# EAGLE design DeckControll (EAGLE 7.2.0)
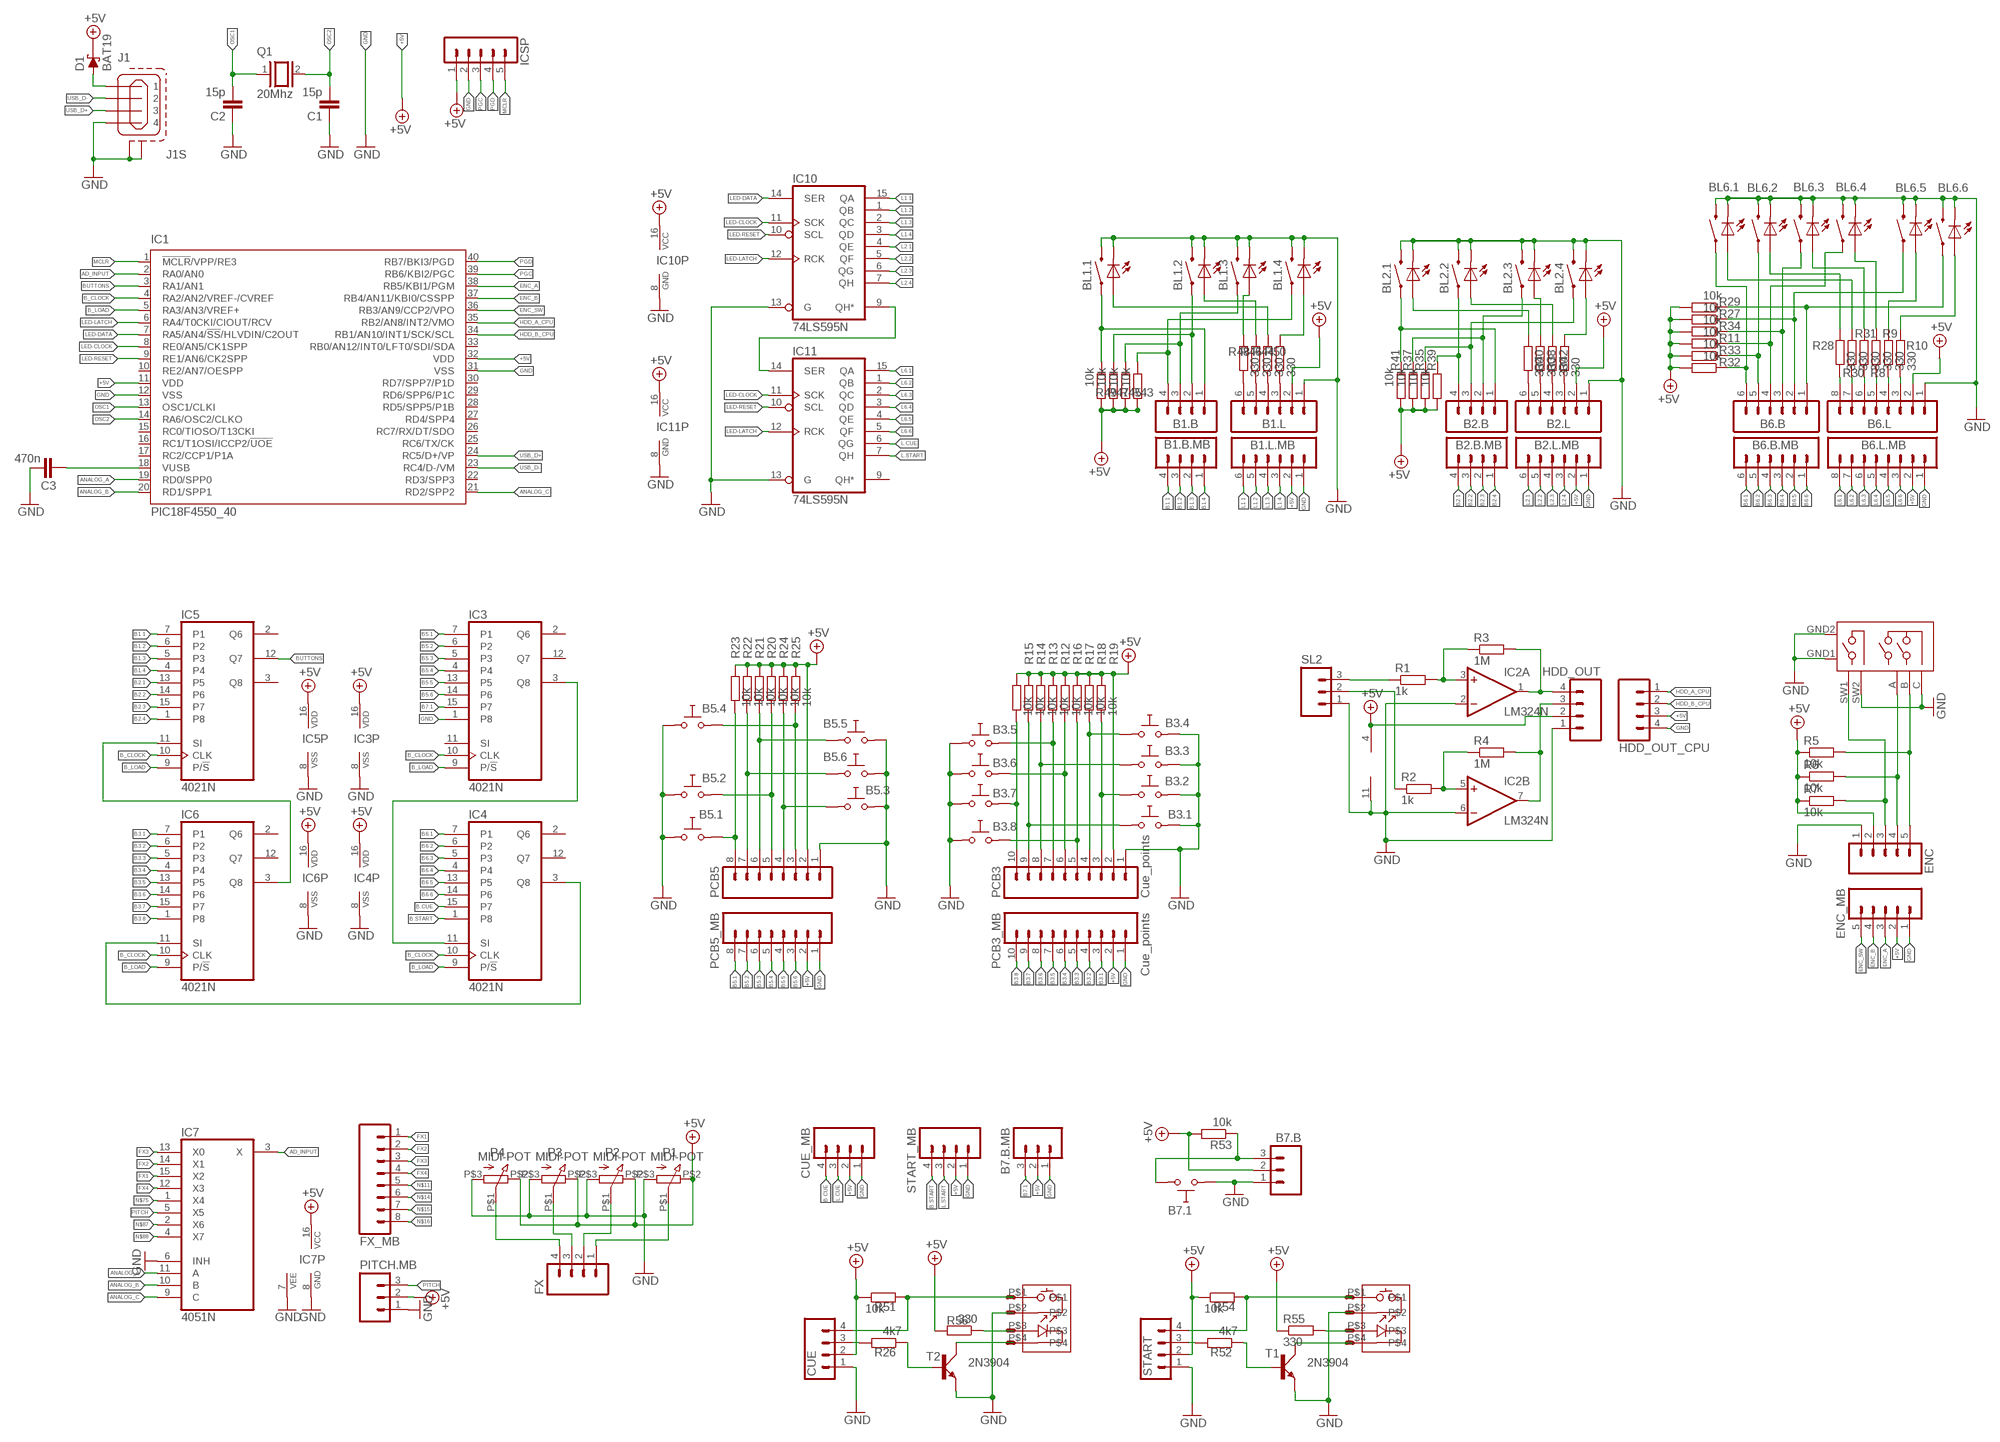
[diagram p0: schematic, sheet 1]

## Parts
ARC01  ARCADE+BTN  [ARCADE_BTN]
ARC02  ARCADE+BTN  [ARCADE_BTN]
B1.B  M04  [04P]
B1.B.MB  M04  [04P]
B1.L  M06  [06P]
B1.L.MB  M06  [06P]
B2.B  M04  [04P]
B2.B.MB  M04  [04P]
B2.L  M06  [06P]
B2.L.MB  M06  [06P]
B3.1  SW-TAKTSS  [SW_TAKT12X12SS]
B3.2  SW-TAKTSS  [SW_TAKT12X12SS]
B3.3  SW-TAKTSS  [SW_TAKT12X12SS]
B3.4  SW-TAKTSS  [SW_TAKT12X12SS]
B3.5  SW-TAKTSS  [SW_TAKT12X12SS]
B3.6  SW-TAKTSS  [SW_TAKT12X12SS]
B3.7  SW-TAKTSS  [SW_TAKT12X12SS]
B3.8  SW-TAKTSS  [SW_TAKT12X12SS]
B5.1  SW-TAKTSS  [SW_TAKT12X12SS]
B5.2  SW-TAKTSS  [SW_TAKT12X12SS]
B5.3  SW-TAKTSS  [SW_TAKT12X12SS]
B5.4  SW-TAKTSS  [SW_TAKT12X12SS]
B5.5  SW-TAKTSS  [SW_TAKT12X12SS]
B5.6  SW-TAKTSS  [SW_TAKT12X12SS]
B6.B  M06  [06P]
B6.B.MB  M06  [06P]
B6.L  M08  [08P]
B6.L.MB  M08  [08P]
B7.1  SW-TAKTSS  [SW_TAKT12X12SS]
B7.B  M03  [03P]
B7.B.MB  M03  [03P]
BL1.1  SWITCH-MOMENTARY-LEDPTH  [TACTILE-PTH-LED-12MM]
BL1.2  SWITCH-MOMENTARY-LEDPTH  [TACTILE-PTH-LED-12MM]
BL1.3  SWITCH-MOMENTARY-LEDPTH  [TACTILE-PTH-LED-12MM]
BL1.4  SWITCH-MOMENTARY-LEDPTH  [TACTILE-PTH-LED-12MM]
BL2.1  SWITCH-MOMENTARY-LEDPTH  [TACTILE-PTH-LED-12MM]
BL2.2  SWITCH-MOMENTARY-LEDPTH  [TACTILE-PTH-LED-12MM]
BL2.3  SWITCH-MOMENTARY-LEDPTH  [TACTILE-PTH-LED-12MM]
BL2.4  SWITCH-MOMENTARY-LEDPTH  [TACTILE-PTH-LED-12MM]
BL6.1  SWITCH-MOMENTARY-LEDPTH  [TACTILE-PTH-LED-12MM]
BL6.2  SWITCH-MOMENTARY-LEDPTH  [TACTILE-PTH-LED-12MM]
BL6.3  SWITCH-MOMENTARY-LEDPTH  [TACTILE-PTH-LED-12MM]
BL6.4  SWITCH-MOMENTARY-LEDPTH  [TACTILE-PTH-LED-12MM]
BL6.5  SWITCH-MOMENTARY-LEDPTH  [TACTILE-PTH-LED-12MM]
BL6.6  SWITCH-MOMENTARY-LEDPTH  [TACTILE-PTH-LED-12MM]
C1  15p  C-EU050-024X044  [C050-024X044]
C2  15p  C-EU050-024X044  [C050-024X044]
C3  470n  C-EU050-024X044  [C050-024X044]
CUE  M04  [04P]
CUE_MB  M04  [04P]
D1  BAT19  [DO35-10]
ENC  M05  [05P]
ENC01  STEC  [STEC]
ENC_MB  M05  [05P]
FX  M04  [04P]
FX_MB  M08  [08P]
HDD_OUT  M04  [04P]
HDD_OUT_CPU  M04  [04P]
IC1  PIC18F4550_40  [DIL40]
IC2  LM324N  [DIL14]
IC3  4021N  [DIL16]
IC4  4021N  [DIL16]
IC5  4021N  [DIL16]
IC6  4021N  [DIL16]
IC7  4051N  [DIL16]
IC10  74LS595N  [DIL16]
IC11  74LS595N  [DIL16]
ICSP  MA05-1  [MA05-1]
J1  MINI-USB_SHIELD4P-85-32004-00X  [85-32004-00X]
P1  MIDI-POT  [MIDI-POT]
P2  MIDI-POT  [MIDI-POT]
P3  MIDI-POT  [MIDI-POT]
P4  MIDI-POT  [MIDI-POT]
PCB3  Cue_points  M10  [10P]
PCB3_MB  Cue_points  M10  [10P]
PCB5  M08  [08P]
PCB5_MB  M08  [08P]
PITCH.MB  M03  [03P]
Q1  20Mhz  XTAL/S  [QS]
R1  1k  R-EU_0207/10  [0207/10]
R2  1k  R-EU_0207/10  [0207/10]
R3  1M  R-EU_0207/10  [0207/10]
R4  1M  R-EU_0207/10  [0207/10]
R5  10k  R-EU_0207/10  [0207/10]
R6  10k  R-EU_0207/10  [0207/10]
R7  10k  R-EU_0207/10  [0207/10]
R8  330  R-EU_0207/10  [0207/10]
R9  330  R-EU_0207/10  [0207/10]
R10  330  R-EU_0207/10  [0207/10]
R11  10k  R-EU_0207/10  [0207/10]
R12  10k  R-EU_0207/10  [0207/10]
R13  10k  R-EU_0207/10  [0207/10]
R14  10k  R-EU_0207/10  [0207/10]
R15  10k  R-EU_0207/10  [0207/10]
R16  10k  R-EU_0207/10  [0207/10]
R17  10k  R-EU_0207/10  [0207/10]
R18  10k  R-EU_0207/10  [0207/10]
R19  10k  R-EU_0207/10  [0207/10]
R20  10k  R-EU_0207/10  [0207/10]
R21  10k  R-EU_0207/10  [0207/10]
R22  10k  R-EU_0207/10  [0207/10]
R23  10k  R-EU_0207/10  [0207/10]
R24  10k  R-EU_0207/10  [0207/10]
R25  10k  R-EU_0207/10  [0207/10]
R26  4k7  R-EU_0207/10  [0207/10]
R27  10k  R-EU_0207/10  [0207/10]
R28  330  R-EU_0207/10  [0207/10]
R29  10k  R-EU_0207/10  [0207/10]
R30  330  R-EU_0207/10  [0207/10]
R31  330  R-EU_0207/10  [0207/10]
R32  10k  R-EU_0207/10  [0207/10]
R33  10k  R-EU_0207/10  [0207/10]
R34  10k  R-EU_0207/10  [0207/10]
R35  10k  R-EU_0207/10  [0207/10]
R36  330  R-EU_0207/10  [0207/10]
R37  10k  R-EU_0207/10  [0207/10]
R38  330  R-EU_0207/10  [0207/10]
R39  10k  R-EU_0207/10  [0207/10]
R40  330  R-EU_0207/10  [0207/10]
R41  10k  R-EU_0207/10  [0207/10]
R42  330  R-EU_0207/10  [0207/10]
R43  10k  R-EU_0207/10  [0207/10]
R44  330  R-EU_0207/10  [0207/10]
R45  10k  R-EU_0207/10  [0207/10]
R46  330  R-EU_0207/10  [0207/10]
R47  10k  R-EU_0207/10  [0207/10]
R48  330  R-EU_0207/10  [0207/10]
R49  10k  R-EU_0207/10  [0207/10]
R50  330  R-EU_0207/10  [0207/10]
R51  10k  R-EU_0207/10  [0207/10]
R52  4k7  R-EU_0207/10  [0207/10]
R53  10k  R-EU_0207/10  [0207/10]
R54  10k  R-EU_0207/10  [0207/10]
R55  330  R-EU_0207/10  [0207/10]
R56  330  R-EU_0207/10  [0207/10]
SL2  M03  [03P]
START  M04  [04P]
START_MB  M04  [04P]
T1  2N3904  [TO92D]
T2  2N3904  [TO92D]

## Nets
+5V: B1.L.2 B1.L.MB.2 B2.L.2 B2.L.MB.2 B6.L.2 B6.L.MB.2 B7.B.2 B7.B.MB.2 CUE.2 CUE_MB.2 D1.C ENC.2 ENC_MB.2 HDD_OUT.2 HDD_OUT_CPU.3 IC1.11(VDD) IC1.32(VDD) IC2.4(P:V+) IC3.16(VDD) IC4.16(VDD) IC5.16(VDD) IC6.16(VDD) IC7.16(VCC) IC10.16(VCC) IC11.16(VCC) ICSP.1 P1.P$2(E) P2.P$2(E) P3.P$2(E) P4.P$2(E) PCB3.2 PCB3_MB.2 PCB5.2 PCB5_MB.2 PITCH.MB.2 R5.1 R6.1 R7.1 R11.2 R12.2 R13.2 R14.2 R15.2 R16.2 R17.2 R18.2 R19.2 R20.2 R21.2 R22.2 R23.2 R24.2 R25.2 R27.2 R29.2 R32.2 R33.2 R34.2 R35.2 R37.2 R39.2 R41.2 R43.2 R45.2 R47.2 R49.2 R51.1 R53.2 R54.1 R55.1 R56.2 START.2 START_MB.2
AD_INPUT: IC1.2(RA0/AN0) IC7.3(X)
ANALOG_A: IC1.19(RD0/SPP0) IC7.11(A)
ANALOG_B: IC1.20(RD1/SPP1) IC7.10(B)
ANALOG_C: IC1.21(RD2/SPP2) IC7.9(C)
B1.1: B1.B.MB.4 IC5.7(P1)
B1.2: B1.B.MB.3 IC5.6(P2)
B1.3: B1.B.MB.2 IC5.5(P3)
B1.4: B1.B.MB.1 IC5.4
B2.1: B2.B.MB.4 IC5.13(P5)
B2.2: B2.B.MB.3 IC5.14(P6)
B2.3: B2.B.MB.2 IC5.15(P7)
B2.4: B2.B.MB.1 IC5.1(P8)
B3.1: IC6.7(P1) PCB3_MB.3
B3.2: IC6.6(P2) PCB3_MB.4
B3.3: IC6.5(P3) PCB3_MB.5
B3.4: IC6.4 PCB3_MB.6
B3.5: IC6.13(P5) PCB3_MB.7
B3.6: IC6.14(P6) PCB3_MB.8
B3.7: IC6.15(P7) PCB3_MB.9
B3.8: IC6.1(P8) PCB3_MB.10
B5.1: IC3.7(P1) PCB5_MB.8
B5.2: IC3.6(P2) PCB5_MB.7
B5.3: IC3.5(P3) PCB5_MB.6
B5.4: IC3.4 PCB5_MB.5
B5.5: IC3.13(P5) PCB5_MB.4
B5.6: IC3.14(P6) PCB5_MB.3
B6.1: B6.B.MB.6 IC4.7(P1)
B6.2: B6.B.MB.5 IC4.6(P2)
B6.3: B6.B.MB.4 IC4.5(P3)
B6.4: B6.B.MB.3 IC4.4
B6.5: B6.B.MB.2 IC4.13(P5)
B6.6: B6.B.MB.1 IC4.14(P6)
B7.1: B7.B.MB.3 IC3.15(P7)
B.CUE: CUE_MB.4 IC4.15(P7)
B.START: IC4.1(P8) START_MB.4
B_CLOCK: IC1.4(RA2/AN2/VREF-/CVREF) IC3.10(CLK) IC4.10(CLK) IC5.10(CLK) IC6.10(CLK)
B_LOAD: IC1.5(RA3/AN3/VREF+) IC3.9(P/!S) IC4.9(P/!S) IC5.9(P/!S) IC6.9(P/!S)
BUTTONS: IC1.3(RA1/AN1) IC5.12(Q7)
ENC_A: ENC_MB.3 IC1.38(RB5/KBI1/PGM)
ENC_A_: ENC01.A ENC.4 R6.2
ENC_B: ENC_MB.4 IC1.37(RB4/AN11/KBI0/CSSPP)
ENC_B_: ENC01.B ENC.5 R5.2
ENC_SW: ENC_MB.5 IC1.36(RB3/AN9/CCP2/VPO)
ENC_SW_: ENC01.SW1 ENC.3 R7.2
FX1: FX_MB.1 IC7.15(X2)
FX2: FX_MB.2 IC7.14(X1)
FX3: FX_MB.3 IC7.13(X0)
FX4: FX_MB.4 IC7.12(X3)
GND: ARC01.P$2 ARC02.P$2 B1.L.1 B1.L.MB.1 B2.L.1 B2.L.MB.1 B3.1.P$1 B3.2.P$1 B3.3.P$1 B3.4.P$1 B3.5.P$1 B3.6.P$1 B3.7.P$1 B3.8.P$1 B5.1.P$1 B5.2.P$1 B5.3.P$2 B5.4.P$1 B5.5.P$2 B5.6.P$2 B6.L.1 B6.L.MB.1 B7.1.P$1 B7.B.1 B7.B.MB.1 BL1.1.2 BL1.1.C BL1.2.2 BL1.2.C BL1.3.2 BL1.3.C BL1.4.2 BL1.4.C BL2.1.2 BL2.1.C BL2.2.2 BL2.2.C BL2.3.2 BL2.3.C BL2.4.2 BL2.4.C BL6.1.2 BL6.1.C BL6.2.2 BL6.2.C BL6.3.2 BL6.3.C BL6.4.2 BL6.4.C BL6.5.2 BL6.5.C BL6.6.2 BL6.6.C C1.1 C2.1 C3.1 CUE.1 CUE_MB.1 ENC01.C(COMMON) ENC01.GND1 ENC01.GND2 ENC01.SW2 ENC.1 ENC_MB.1 HDD_OUT.1 HDD_OUT_CPU.4 IC1.12(VSS) IC1.31(VSS) IC2.2(A:-IN) IC2.6(B:-IN) IC2.11(P:V-) IC3.1(P8) IC3.8(VSS) IC4.8(VSS) IC5.8(VSS) IC6.8(VSS) IC7.6(INH) IC7.7(VEE) IC7.8(GND) IC10.8(GND) IC10.13(G) IC11.8(GND) IC11.13(G) ICSP.2 J1.4 J1.M1(S1) J1.M2(S2) P1.P$3(A) P2.P$3(A) P3.P$3(A) P4.P$3(A) PCB3.1 PCB3_MB.1 PCB5.1 PCB5_MB.1 PITCH.MB.1 SL2.1 START.1 START_MB.1 T1.E T2.E
HDD_A_CPU: HDD_OUT_CPU.1 IC1.35(RB2/AN8/INT2/VMO)
HDD_B_CPU: HDD_OUT_CPU.2 IC1.34(RB1/AN10/INT1/SCK/SCL)
L1.1: B1.L.MB.6 IC10.15(QA)
L1.2: B1.L.MB.5 IC10.1(QB)
L1.3: B1.L.MB.4 IC10.2(QC)
L1.4: B1.L.MB.3 IC10.3(QD)
L2.1: B2.L.MB.6 IC10.4(QE)
L2.2: B2.L.MB.5 IC10.5(QF)
L2.3: B2.L.MB.4 IC10.6(QG)
L2.4: B2.L.MB.3 IC10.7(QH)
L6.1: B6.L.MB.8 IC11.15(QA)
L6.2: B6.L.MB.7 IC11.1(QB)
L6.3: B6.L.MB.6 IC11.2(QC)
L6.4: B6.L.MB.5 IC11.3(QD)
L6.5: B6.L.MB.4 IC11.4(QE)
L6.6: B6.L.MB.3 IC11.5(QF)
L.CUE: CUE_MB.3 IC11.6(QG)
L.START: IC11.7(QH) START_MB.3
LED-CLOCK: IC1.8(RE0/AN5/CK1SPP) IC10.11(SCK) IC11.11(SCK)
LED-DATA: IC1.7(RA5/AN4/!SS!/HLVDIN/C2OUT) IC10.14(SER)
LED-LATCH: IC1.6(RA4/T0CKI/CIOUT/RCV) IC10.12(RCK) IC11.12(RCK)
LED-RESET: IC1.9(RE1/AN6/CK2SPP) IC10.10(SCL) IC11.10(SCL)
LED.SER: IC10.9(QH*) IC11.14(SER)
MCLR: IC1.1(!MCLR!/VPP/RE3) ICSP.5
N$1: IC5.11(SI) IC6.3(Q8)
N$2: ARC01.P$3 R56.1
N$3: R52.1 T1.B
N$4: CUE.3 R26.2
N$5: C3.2 IC1.18(VUSB)
N$6: R52.2 START.3
N$7: R1.1 SL2.3
N$8: IC2.3(A:+IN) R1.2 R3.1
N$9: IC2.5(B:+IN) R2.2 R4.1
N$10: R2.1 SL2.2
N$11: FX_MB.5
N$12: HDD_OUT.4 IC2.1(A:OUT) R3.2
N$13: HDD_OUT.3 IC2.7(B:OUT) R4.2
N$14: FX_MB.6
N$15: FX_MB.7
N$16: FX_MB.8
N$17: IC4.3(Q8) IC6.11(SI)
N$18: IC3.3(Q8) IC4.11(SI)
N$20: B7.1.P$2 B7.B.3 R53.1
N$21: B6.L.8 R28.1
N$22: B6.B.5 BL6.2.4 R33.1
N$23: B1.L.6 R48.1
N$24: ARC01.P$1 CUE.4 R51.2
N$25: B6.B.3 BL6.3.4 R34.1
N$26: ARC02.P$1 R54.2 START.4
N$27: B1.L.4 R44.1
N$28: B2.L.5 R40.1
N$29: D1.A J1.1
N$30: B6.B.4 BL6.4.4 R11.1
N$31: B6.B.2 BL6.5.4 R27.1
N$32: FX.3 P3.P$1(S)
N$33: B6.L.7 R30.1
N$34: B6.B.1 BL6.6.4 R29.1
N$35: B6.B.6 BL6.1.4 R32.1
N$36: B6.L.4 R9.1
N$37: B6.L.6 R31.1
N$38: B6.L.5 R8.1
N$39: B6.L.3 R10.1
N$40: B2.B.3 BL2.4.4 R35.1
N$41: B2.B.2 BL2.3.4 R37.1
N$42: B2.B.4 BL2.2.4 R39.1
N$43: B2.B.1 BL2.1.4 R41.1
N$44: B2.L.6 R36.1
N$45: B2.L.4 R38.1
N$46: B2.L.3 R42.1
N$47: ARC02.P$3 R55.2
N$48: B1.L.5 R46.1
N$49: R26.1 T2.B
N$50: B1.L.3 R50.1
N$51: B1.B.1 BL1.1.4 R49.1
N$52: B1.B.2 BL1.2.4 R47.1
N$53: FX.4 P4.P$1(S)
N$54: FX.2 P2.P$1(S)
N$55: B1.B.3 BL1.3.4 R45.1
N$56: B1.B.4 BL1.4.4 R43.1
N$57: FX.1 P1.P$1(S)
N$58: B3.5.P$2 PCB3.7 R12.1
N$59: ARC01.P$4 T2.C
N$60: ARC02.P$4 T1.C
N$61: B3.3.P$2 PCB3.8 R13.1
N$62: B3.1.P$2 PCB3.9 R14.1
N$65: B3.7.P$2 PCB3.10 R15.1
N$66: B5.2.P$2 PCB5.5 R20.1
N$67: B3.8.P$2 PCB3.5 R17.1
N$68: B3.4.P$2 PCB3.4 R18.1
N$69: B3.6.P$2 PCB3.6 R16.1
N$70: B3.2.P$2 PCB3.3 R19.1
N$71: B5.3.P$1 PCB5.4 R24.1
N$72: BL6.4.A R8.2
N$73: BL6.5.A R9.2
N$74: BL6.6.A R10.2
N$75: IC7.1(X4)
N$77: BL2.1.A R36.2
N$78: BL2.2.A R38.2
N$79: B5.5.P$1 PCB5.6 R21.1
N$80: B5.6.P$1 PCB5.7 R22.1
N$81: B5.1.P$2 PCB5.8 R23.1
N$82: BL6.1.A R30.2
N$83: B5.4.P$2 PCB5.3 R25.1
N$84: BL2.3.A R40.2
N$85: BL6.2.A R28.2
N$86: BL2.4.A R42.2
N$87: IC7.2(X6)
N$88: IC7.4(X7)
N$94: BL6.3.A R31.2
N$108: BL1.1.A R44.2
N$109: BL1.2.A R46.2
N$110: BL1.3.A R48.2
N$111: BL1.4.A R50.2
OSC1: C2.2 IC1.13(OSC1/CLKI) Q1.1
OSC2: C1.2 IC1.14(RA6/OSC2/CLKO) Q1.2
PGC: IC1.39(RB6/KBI2/PGC) ICSP.3
PGD: IC1.40(RB7/BKI3/PGD) ICSP.4
PITCH: IC7.5(X5) PITCH.MB.3
USB_D+: IC1.24(RC5/D+/VP) J1.3
USB_D-: IC1.23(RC4/D-/VM) J1.2
Unconnected: IC1.10(RE2/AN7/OESPP) IC1.15(RC0/TIOSO/T13CKI) IC1.16(RC1/T1OSI/ICCP2/!UOE) IC1.17(RC2/CCP1/P1A) IC1.22(RD3/SPP3) IC1.25(RC6/TX/CK) IC1.26(RC7/RX/DT/SDO) IC1.27(RD4/SPP4) IC1.28(RD5/SPP5/P1B) IC1.29(RD6/SPP6/P1C) IC1.30(RD7/SPP7/P1D) IC1.33(RB0/AN12/INT0/LFT0/SDI/SDA) IC2.8(C:OUT) IC2.9(C:-IN) IC2.10(C:+IN) IC2.12(D:+IN) IC2.13(D:-IN) IC2.14(D:OUT) IC3.2(Q6) IC3.11(SI) IC3.12(Q7) IC4.2(Q6) IC4.12(Q7) IC5.2(Q6) IC5.3(Q8) IC6.2(Q6) IC6.12(Q7) IC11.9(QH*)

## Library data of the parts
ARC01 ARC02 = w-switches:ARCADE+BTN
B1.B B1.B.MB B2.B B2.B.MB CUE CUE_MB FX HDD_OUT HDD_OUT_CPU START START_MB = con-amp-quick:M04: AMP QUICK CONNECTOR; OC_FARNELL: unknown; OC_NEWARK: unknown
B1.L B1.L.MB B2.L B2.L.MB B6.B B6.B.MB = con-amp-quick:M06: AMP QUICK CONNECTOR; OC_FARNELL: unknown; OC_NEWARK: unknown
B3.1-B3.8 B5.1-B5.6 B7.1 = gogo:SW-TAKT
B6.L B6.L.MB FX_MB PCB5 PCB5_MB = con-amp-quick:M08: AMP QUICK CONNECTOR; OC_FARNELL: unknown; OC_NEWARK: unknown
B7.B B7.B.MB PITCH.MB SL2 = con-amp-quick:M03: AMP QUICK CONNECTOR; OC_FARNELL: unknown; OC_NEWARK: unknown
BL1.1-BL1.4 BL2.1-BL2.4 BL6.1-BL6.6 = Local Library:SWITCH-MOMENTARY-LED
C1-C3 = resistor:C-EU: CAPACITOR, European symbol
D1 = diode:BAT19: DIODE
ENC ENC_MB = con-amp-quick:M05: AMP QUICK CONNECTOR; OC_FARNELL: unknown; OC_NEWARK: unknown
ENC01 = rotary-encoder-STUC:STEC
IC1 = microchip:PIC18F4*_40: USB Microcontrollers with nanoWatt Technology High-Performance, Enhanced Flash, 28/40/44-Pin, Source: http://ww1.microchip.com/downloads/en/devicedoc/39632c.pdf; MF: MICROCHIP; MPN: PIC18F4550-I/P; OC_FARNELL: 9321357; OC_NEWARK: 74K8623
IC2 = linear:LM324: OP AMP
IC3-IC6 = 40xx:4021: 8-bit static SHIFT REGISTER
IC7 = 40xx:4051: 8-channel ANALOG MULTIPLEXER
IC10 IC11 = 74xx-eu:74*595: 8-bit SHIFT REGISTER, output latch
ICSP = con-lstb:MA05-1: PIN HEADER; OC_FARNELL: unknown; OC_NEWARK: unknown
J1 = con-cypressindustries:MINI-USB_SHIELD4P-: MINI USB 4 Pol. Source: www.cypressindustries.com
P1-P4 = pot:MIDI-POT
PCB3 PCB3_MB = con-amp-quick:M10: AMP QUICK CONNECTOR; OC_FARNELL: unknown; OC_NEWARK: unknown
Q1 = special:XTAL/S: CRYSTAL
R1-R56 = rcl:R-EU_: RESISTOR, European symbol
T1 T2 = transistor-small-signal:2N3904: NPN TRANSISTOR

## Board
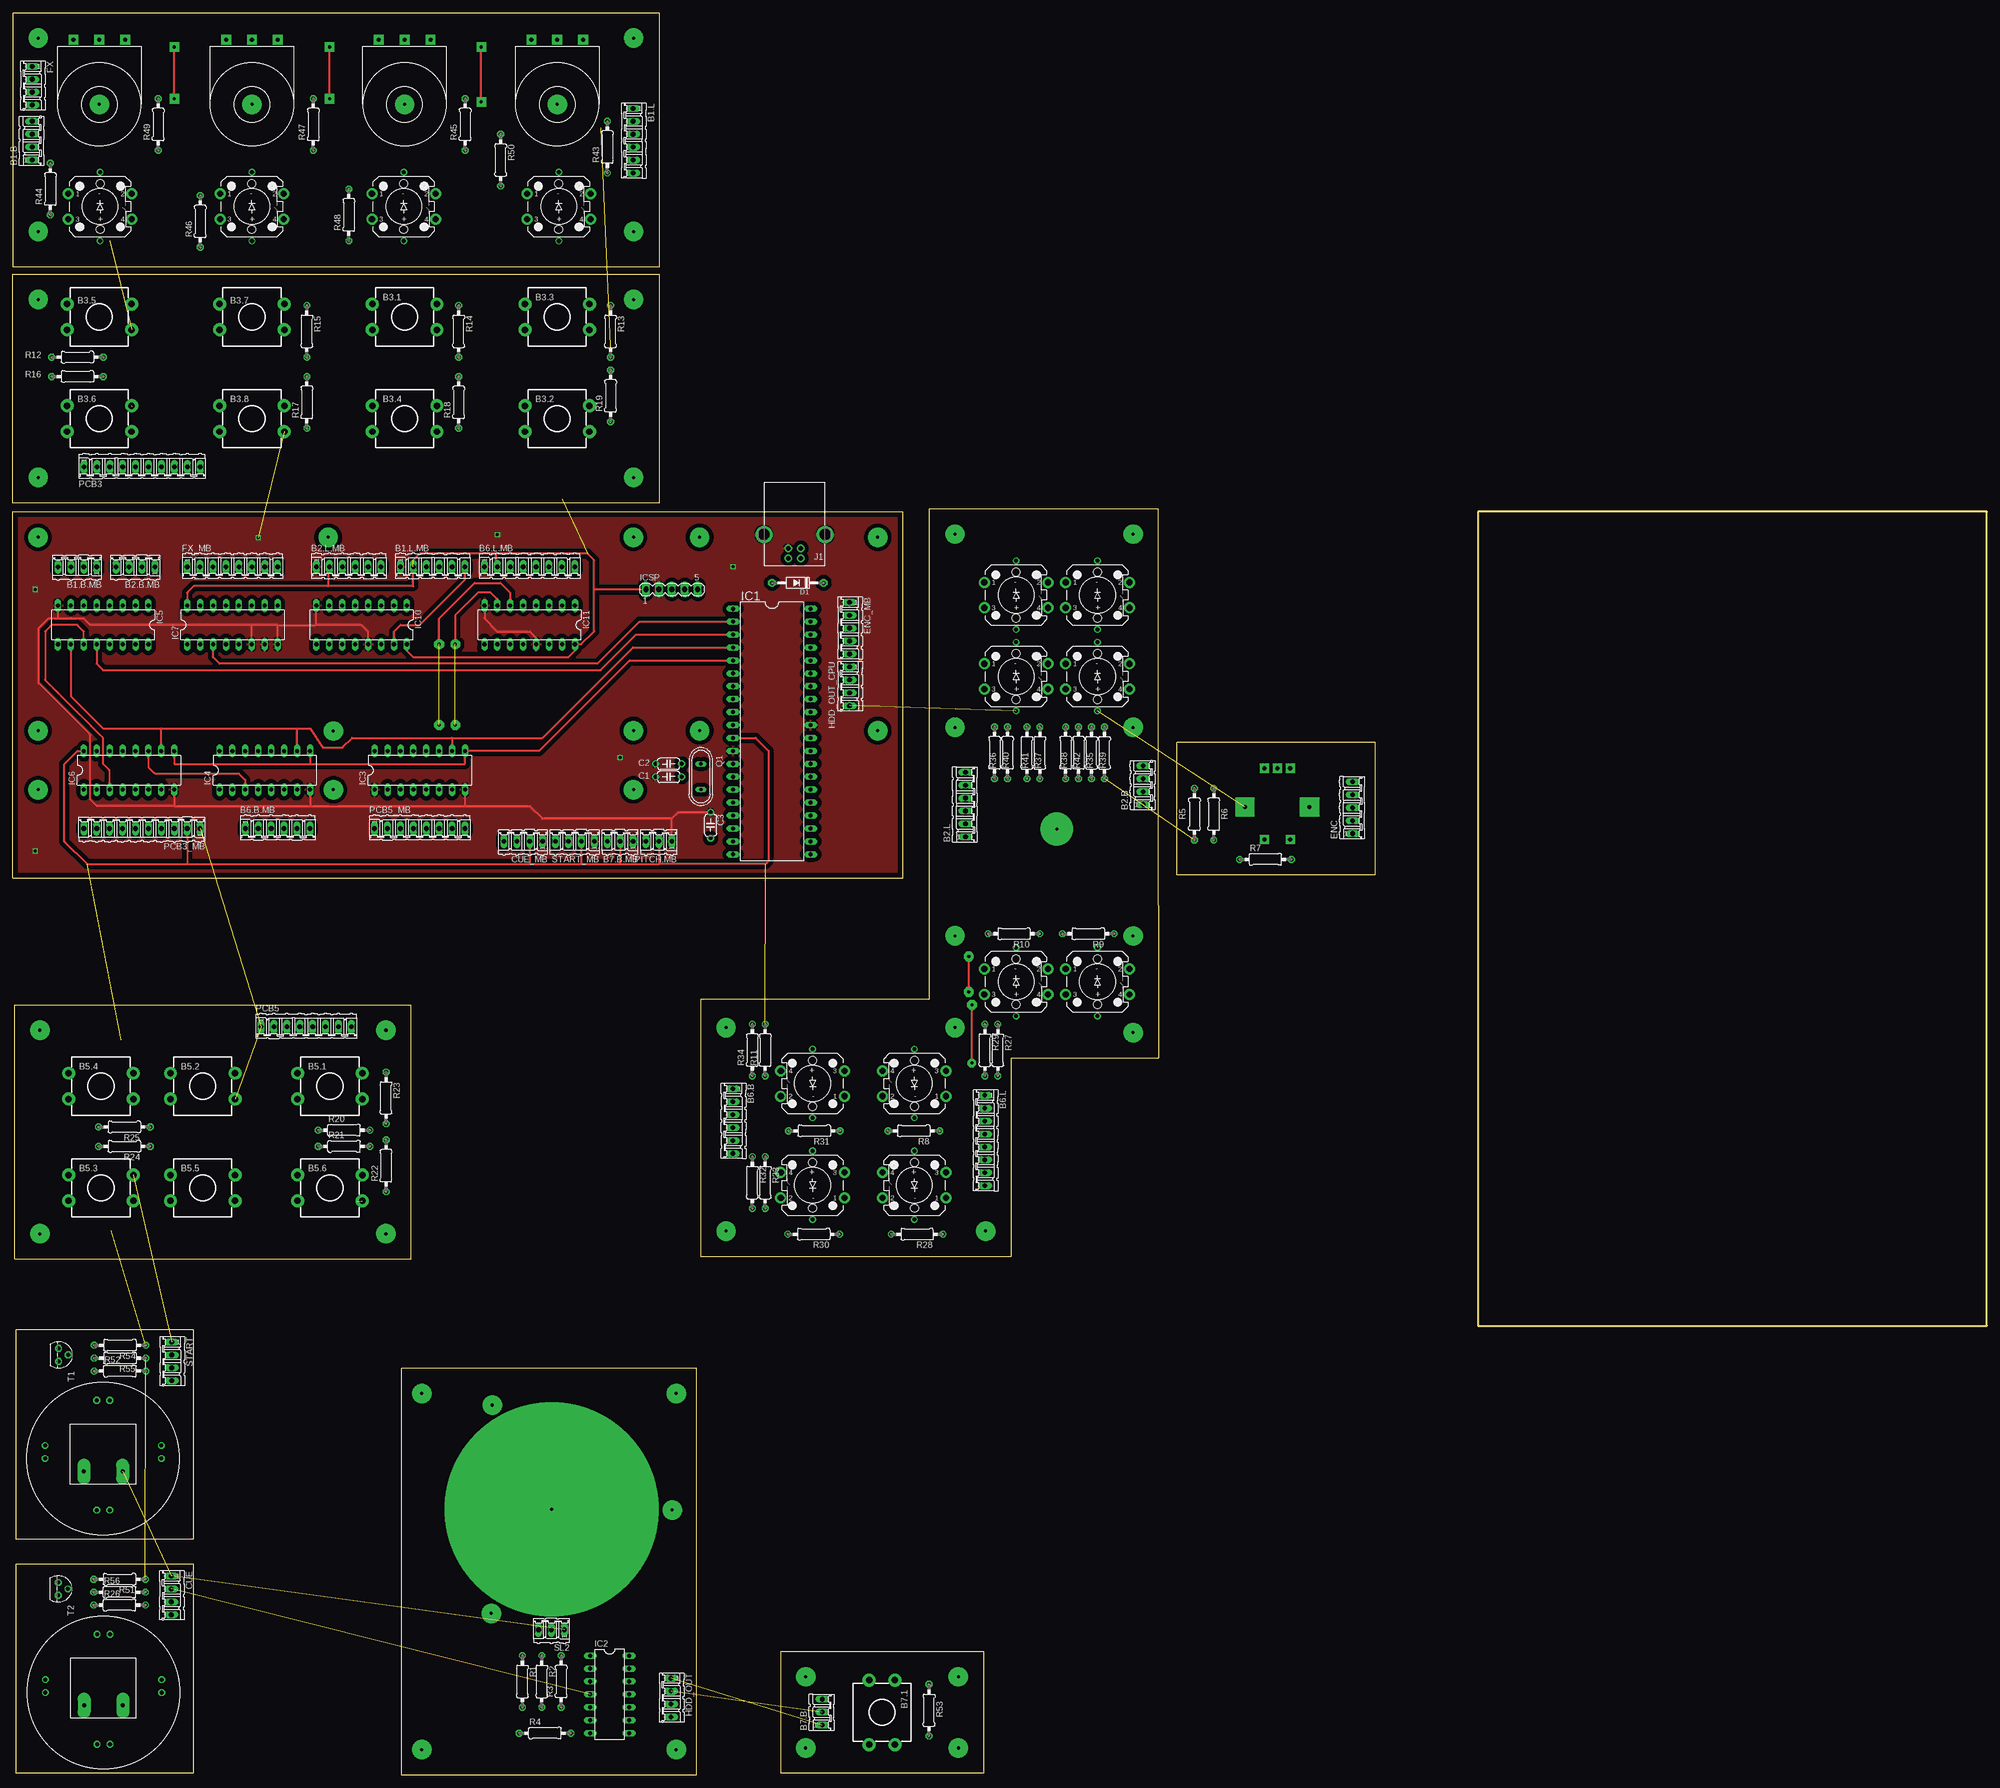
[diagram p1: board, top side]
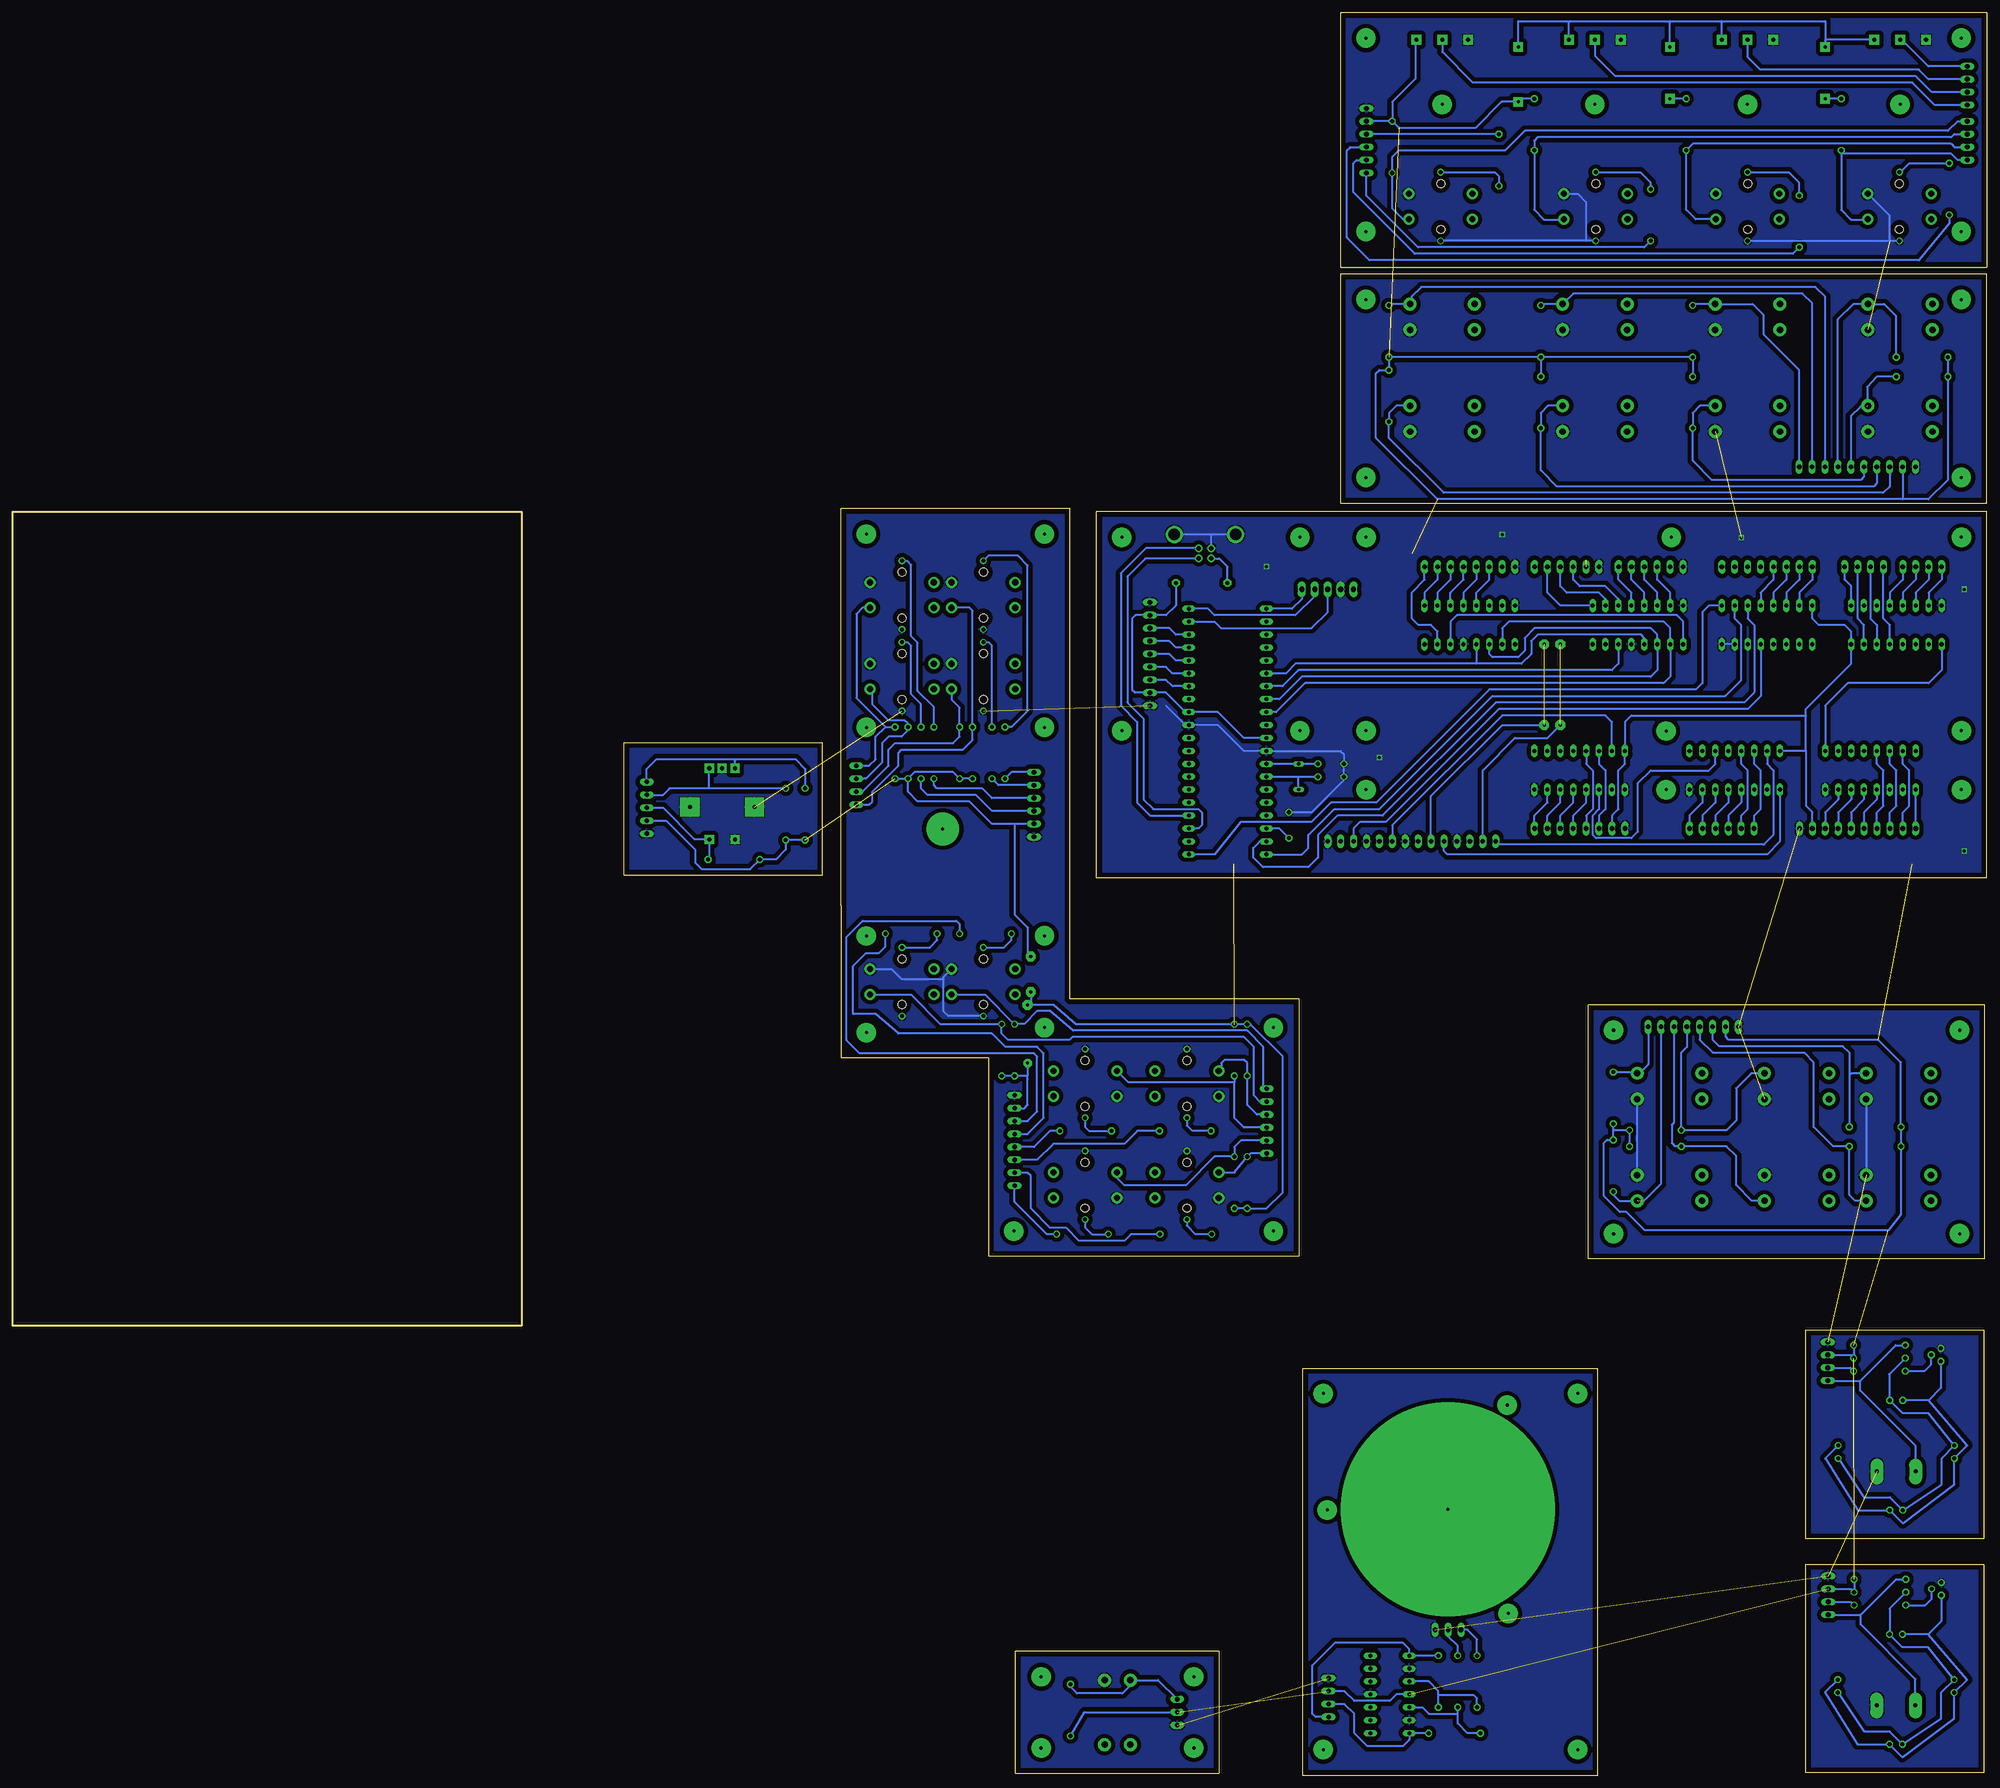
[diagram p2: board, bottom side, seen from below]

Size 388 x 346.41 mm. Coordinates in mm from the lower left corner, seen from the top.
Outline: 50 segments
Copper layers (1*16): Top 0.035mm / dielectric 1.5mm / Bottom 0.035mm
Design rules "default": minimum track width 10mil, minimum drill 24mil, track to track 8mil, track to pad 8mil, pad to pad 8mil, via to via 8mil, smd to smd 8mil, copper to edge 40mil, drill to drill 8mil, minimum pad ring 10mil, minimum via ring 8mil, stop-mask expansion 4mil, vias tented up to drill 0mil, thermal gap 10mil

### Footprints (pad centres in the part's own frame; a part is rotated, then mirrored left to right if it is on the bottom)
ARCADE_BTN = drill 0.8 pad 2.54 long: P$1 3.81,2.54; P$2 -3.81,2.54 | drill 0.8 octagon: P$3 -11.43,0; P$4 -11.43,-2.54; P$5 -1.27,10.16; P$6 1.27,10.16; P$7 11.43,0; P$8 11.43,-2.54; P$9 -1.27,-11.43; P$10 1.27,-11.43
04P = drill 0.914 long: 1 -3.81,0; 2 -1.27,0; 3 1.27,0; 4 3.81,0
06P = drill 0.914 long: 1 -6.35,0; 2 -3.81,0; 3 -1.27,0; 4 1.27,0; 5 3.81,0; 6 6.35,0
SW_TAKT12X12SS = drill 1.27 pad 2.54: P$1 -2.54,-6.35; P$2 2.54,-6.35; P$3 2.54,6.35; P$4 -2.54,6.35
08P = drill 0.914 long: 1 -8.89,0; 2 -6.35,0; 3 -3.81,0; 4 -1.27,0; 5 1.27,0; 6 3.81,0; 7 6.35,0; 8 8.89,0
03P = drill 0.914 long: 1 -2.54,0; 2 0,0; 3 2.54,0
TACTILE-PTH-LED-12MM = drill 1.2 pad 2.159: 1 -6.25,2.5; 2 6.25,2.5; 3 -6.25,-2.5; 4 6.25,-2.5 | drill 0.8: A 0,6.75; C 0,-6.75 | hole 1.6: 0,4.5; 0,-4.5
C050-024X044 = drill 0.813 octagon: 1 -2.54,0; 2 2.54,0
DO35-10 = drill 0.813 pad 1.524 octagon: A 5.08,0; C -5.08,0
05P = drill 0.914 long: 1 -5.08,0; 2 -2.54,0; 3 0,0; 4 2.54,0; 5 5.08,0
STEC = drill 0.8 pad 1.778 square: A -2.54,-7.62; B 2.54,-7.62; C 0,-7.62; SW1 -2.54,6.35; SW2 2.54,6.35 | drill 0.8 pad 3.81 square: GND1 -6.35,0; GND2 6.35,0
DIL40 = drill 0.813 long: 1 -24.13,-7.62; 2 -21.59,-7.62; 3 -19.05,-7.62; 4 -16.51,-7.62; 5 -13.97,-7.62; 6 -11.43,-7.62; 7 -8.89,-7.62; 8 -6.35,-7.62; 9 -3.81,-7.62; 10 -1.27,-7.62; 11 1.27,-7.62; 12 3.81,-7.62; 13 6.35,-7.62; 14 8.89,-7.62; 15 11.43,-7.62; 16 13.97,-7.62; 17 16.51,-7.62; 18 19.05,-7.62; 19 21.59,-7.62; 20 24.13,-7.62; 21 24.13,7.62; 22 21.59,7.62; 23 19.05,7.62; 24 16.51,7.62; 25 13.97,7.62; 26 11.43,7.62; 27 8.89,7.62; 28 6.35,7.62; 29 3.81,7.62; 30 1.27,7.62; 31 -1.27,7.62; 32 -3.81,7.62; 33 -6.35,7.62; 34 -8.89,7.62; 35 -11.43,7.62; 36 -13.97,7.62; 37 -16.51,7.62; 38 -19.05,7.62; 39 -21.59,7.62; 40 -24.13,7.62
DIL14 = drill 0.813 long: 1 -7.62,-3.81; 2 -5.08,-3.81; 3 -2.54,-3.81; 4 0,-3.81; 5 2.54,-3.81; 6 5.08,-3.81; 7 7.62,-3.81; 8 7.62,3.81; 9 5.08,3.81; 10 2.54,3.81; 11 0,3.81; 12 -2.54,3.81; 13 -5.08,3.81; 14 -7.62,3.81
DIL16 = drill 0.813 long: 1 -8.89,-3.81; 2 -6.35,-3.81; 3 -3.81,-3.81; 4 -1.27,-3.81; 5 1.27,-3.81; 6 3.81,-3.81; 7 6.35,-3.81; 8 8.89,-3.81; 9 8.89,3.81; 10 6.35,3.81; 11 3.81,3.81; 12 1.27,3.81; 13 -1.27,3.81; 14 -3.81,3.81; 15 -6.35,3.81; 16 -8.89,3.81
MA05-1 = drill 1.016 long: 1 -5.08,0; 2 -2.54,0; 3 0,0; 4 2.54,0; 5 5.08,0
85-32004-00X = drill 0.92 pad 1.27: 1 4.71,-1.25; 2 4.71,1.25; 3 2.71,1.25; 4 2.71,-1.25 | drill 2.3 pad 3: M1 0,6.02; M2 0,-6.02
MIDI-POT = drill 0.8 pad 1.93 square: P$1 0,12.7; P$2 5.08,12.7; P$3 -5.08,12.7
10P = drill 0.914 long: 1 -11.43,0; 2 -8.89,0; 3 -6.35,0; 4 -3.81,0; 5 -1.27,0; 6 1.27,0; 7 3.81,0; 8 6.35,0; 9 8.89,0; 10 11.43,0
QS = drill 0.61 long: 1 -2.54,0; 2 2.54,0
0207/10 = drill 0.813 octagon: 1 -5.08,0; 2 5.08,0
TO92D = drill 0.813 octagon: B 0,1.905; C 1.27,0; E -1.27,0

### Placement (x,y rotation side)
ARC01  17.85,16.24 180 top
ARC02  17.78,62.24 180 top
B1.B  3.83,321.26 90 top
B1.B.MB  12.7,237.51 180 top
B1.L  121.94,321.26 270 top
B1.L.MB  82.55,237.51 0 top
B2.B  222.19,194.59 90 top
B2.B.MB  24.13,237.51 180 top
B2.L  187.27,190.78 90 top
B2.L.MB  66.04,237.51 0 top
B3.1  77.03,286.62 90 top
B3.2  107.03,266.62 90 top
B3.3  107.03,286.62 90 top
B3.4  77.03,266.62 90 top
B3.5  17.02,286.62 90 top
B3.6  17.02,266.62 90 top
B3.7  47.02,286.62 90 top
B3.8  47.02,266.62 90 top
B5.1  62.35,135.42 90 top
B5.2  37.35,135.42 90 top
B5.3  17.35,115.42 90 top
B5.4  17.35,135.42 90 top
B5.5  37.35,115.42 90 top
B5.6  62.35,115.42 90 top
B6.B  141.55,128.55 270 top
B6.B.MB  52.07,186.08 0 top
B6.L  191.08,124.74 270 top
B6.L.MB  101.6,237.51 0 top
B7.1  170.87,12.33 180 top
B7.B  159.1,12.37 90 top
B7.B.MB  119.38,183.53 180 top
BL1.1  17.17,308.31 0 top
BL1.2  47.01,308.31 0 top
BL1.3  76.86,308.31 0 top
BL1.4  107.34,308.31 0 top
BL2.1  197.21,231.94 0 top
BL2.2  213.21,231.94 0 top
BL2.3  197.21,215.94 0 top
BL2.4  213.21,215.94 0 top
BL6.1  157.21,115.94 180 top
BL6.2  177.21,115.94 180 top
BL6.3  157.21,135.94 180 top
BL6.4  177.21,135.94 180 top
BL6.5  213.21,155.94 0 top
BL6.6  197.21,155.94 0 top
C1  128.91,196.24 0 top
C2  128.91,198.78 0 top
C3  137.16,186.71 270 top
CUE  31.16,35.33 270 top
CUE_MB  100.33,183.53 180 top
D1  154.31,234.34 180 top
ENC  263.37,190.15 90 top
ENC01  248.55,190.28 180 top
ENC_MB  164.47,225.44 270 top
FX  3.83,332.06 270 top
FX_MB  43.18,237.51 0 top
HDD_OUT  129.38,15.24 270 top
HDD_OUT_CPU  164.47,214.02 270 top
IC1  149.22,205.12 270 top
IC2  117.32,15.87 270 top
IC3  80.01,197.5 0 top
IC4  49.53,197.5 0 top
IC5  17.78,226.08 180 top
IC6  22.86,197.5 0 top
IC7  43.18,226.08 0 top
IC10  68.58,226.08 180 top
IC11  101.6,226.08 180 top
ICSP  129.54,233.06 0 top
J1  153.67,243.86 270 top
P1  17.02,328.41 0 top
P2  47.02,328.41 0 top
P3  77.02,328.41 0 top
P4  107.02,328.41 0 top
PCB3  25.43,257.12 0 top
PCB3_MB  25.4,186.08 180 top
PCB5  57.68,147.08 0 top
PCB5_MB  80.01,186.08 0 top
PITCH.MB  127,183.53 180 top
Q1  135.25,196.24 270 top
R1  100.17,18.41 270 top
R2  103.98,18.41 270 top
R3  107.8,18.41 90 top
R4  104.62,8.25 0 top
R5  232.26,188.88 90 top
R6  236.07,188.88 90 top
R7  246.23,179.99 0 top
R8  177.11,126.64 180 top
R9  211.4,165.38 180 top
R10  196.79,165.38 180 top
R11  147.9,142.52 90 top
R12  12.72,278.71 180 top
R13  117.5,283.79 270 top
R14  87.66,283.79 270 top
R15  57.81,283.79 270 top
R16  12.72,274.9 180 top
R17  57.81,269.82 90 top
R18  87.66,269.82 90 top
R19  117.5,271.09 90 top
R20  65.12,126.76 0 top
R21  65.12,123.58 0 top
R22  73.38,119.77 90 top
R23  73.38,133.11 270 top
R24  21.94,123.58 180 top
R25  21.94,127.39 180 top
R26  21,33.42 0 top
R27  193.62,142.52 270 top
R28  177.74,106.32 180 top
R29  191.08,142.52 270 top
R30  157.42,106.32 180 top
R31  157.54,126.64 180 top
R32  145.36,116.48 270 top
R33  147.9,116.48 270 top
R34  145.36,142.52 90 top
R35  212.03,200.94 270 top
R36  192.98,200.94 90 top
R37  201.87,200.94 270 top
R38  206.95,200.94 90 top
R39  214.57,200.94 270 top
R40  195.52,200.94 90 top
R41  199.33,200.94 270 top
R42  209.49,200.94 90 top
R43  116.86,319.99 90 top
R44  7.39,311.74 90 top
R45  88.92,324.44 90 top
R46  36.85,305.39 90 top
R47  59.08,324.44 90 top
R48  66.06,306.66 90 top
R49  28.6,324.44 90 top
R50  95.91,317.45 270 top
R51  21,38.5 180 top
R52  21.09,79.42 0 top
R53  180.09,12.76 270 top
R54  21.09,84.5 180 top
R55  21.09,81.96 180 top
R56  21,35.96 0 top
SL2  105.89,28.57 180 top
START  31.25,81.33 270 top
START_MB  110.49,183.53 180 top
T1  9.02,82.6 270 top
T2  8.94,36.6 270 top

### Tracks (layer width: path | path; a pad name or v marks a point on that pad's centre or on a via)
+5V  (via drill 0.6 pad 1.68, 0.6 pad 1.93)  (10 unrouted)
  Top 0.406: PITCH.MB.2 127,179.09 | 62,233.7 78.74,233.7 B1.L.MB.2 | 62,233.7 35.56,233.7 34.29,232.43 IC7.16 | IC10.16 77.47,221 78.74,219.73 109.22,219.73 110.49,221 IC11.16 111.76,222.27 114.3,224.81 114.3,233.06 | 78.74,238.78 80.01,240.05 95,240.05 | 114.3,233.06 114.3,238.78 113.03,240.05 95,240.05 | IC1.11 146.05,203.86 148.59,201.31 148.59,179.72 147.96,179.09 127,179.09 | 34.29,179.09 14.61,179.09 10.16,183.53 10.16,198.78 12.7,201.31 IC6.16 | 34.29,179.09 101.6,179.09 | 101.6,179.09 111.76,179.09 | 111.76,179.09 119.38,179.09 | 119.38,179.09 127,179.09 | ICSP.1 114.3,233.06 | v188.54,139.98 v188.54,151.41 | v187.9,160.93 v187.9,153.95 | v31.77,329.52 v31.77,339.68 | v62.26,329.52 v62.26,339.68 | v92.1,328.88 v92.1,339.68 | PCB3_MB.2 34.29,179.09 | B6.L.MB.2 95,237.76 95,240.05 | B2.L.MB.2 62,237.28 62,233.7 | B7.B.MB.2 119.38,179.09 | START_MB.2 111.76,179.09 | CUE_MB.2 101.6,179.09
  Bottom 0.406: IC7.16 34.29,227.35 33.02,226.08 27.94,226.08 26.67,224.81 IC5.16 26.67,218.46 35.56,209.57 35.56,208.3 | 35.56,201.31 35.56,208.3 | 35.56,208.3 69.85,208.3 71.12,207.03 IC3.16 71.12,198.78 72.39,197.5 72.39,189.89 73.66,188.62 PCB5_MB.2 | 35.56,201.31 IC4.16 | IC1.11 146.05,203.86 151.13,208.94 IC1.32 157.48,208.94 161.29,212.75 HDD_OUT_CPU.3 167.44,212.75 168,213.31 168,227.31 167.32,227.99 ENC_MB.2 161.29,227.99 159.38,229.89 D1.C | R14.2 R15.2 R17.2 | R14.2 R13.2 R19.2 119.41,276.17 120.04,275.54 120.04,262.84 107.97,250.77 16.54,250.77 | R12.2 R16.2 7.64,254.58 11.46,250.77 16.54,250.77 | R14.2 R18.2 | R21.2 R20.2 73.38,126.76 | PCB5.2 51.33,145.17 50.69,144.54 21.31,144.54 16.86,140.09 R25.2 R24.2 16.86,110.25 19.4,107.07 67.21,107.07 70.83,110.7 72.11,110.7 75.28,113.87 75.28,124.22 74.65,124.85 R22.2 73.38,126.76 | 73.38,126.76 R23.2 | P4.P$2 112.26,340.95 112.26,333.49 116.86,328.88 R43.2 | R43.2 B1.L.2 | PCB3.2 16.54,250.77 | R5.1 R6.1 236.07,181.9 237.97,179.99 R7.1 243.05,178.09 252.58,178.09 253.85,179.36 253.85,181.9 259.56,187.61 ENC.2 | R33.2 R32.2 141.55,111.4 138.37,114.58 138.37,141.25 144.72,147.6 R34.2 R11.2 179.01,147.6 183.46,151.41 187.84,151.41 | R27.2 R29.2 188.54,137.44 | R41.2 R37.2 203.14,197.13 210.76,197.13 R35.2 | R39.2 R35.2 | 191.08,186.97 195.52,186.97 199.97,191.41 210.13,191.41 212.03,193.32 R35.2 | B6.L.2 189.17,131.09 188.54,131.72 188.54,136.8 188.54,137.44 | 187.84,151.41 v188.54,151.41 | B2.L.2 191.08,186.97 | 191.08,186.97 191.08,169.19 188.54,166.65 188.54,161.57 v187.9,160.93 | R53.2 177.3,12.37 B7.B.2 | IC2.4 116.05,15.87 117.32,14.6 124.31,14.6 126.21,16.5 HDD_OUT.2
  Bottom 0.406: CUE.2 26.72,36.6 R56.2 R51.1 | START.2 26.17,82.6 R55.1 R54.1 | R49.2 v31.77,329.52 | P1.P$2 31.61,341.11 31.77,340.95 | R47.2 v62.26,329.52 | 81.94,344.76 92.1,344.76 v92.1,339.68 | 81.94,344.76 62.26,344.76 | 62.26,344.76 52.09,344.76 | 52.09,344.76 31.77,344.76 31.77,340.95 | 31.77,340.95 v31.77,339.68 | v62.26,339.68 62.26,344.76 | P3.P$2 82.1,344.6 81.94,344.76 | P2.P$2 52.1,344.75 52.09,344.76 | R43.2 115.59,323.8 100.44,323.8 95.36,328.88 v92.1,328.88 91.47,329.52 R45.2 | v188.54,139.98 188.54,137.44 | v187.9,153.95 187.9,151.47 187.84,151.41 | PCB3_MB.2 34.29,189.27 35.56,190.53 35.56,201.31
AD_INPUT
  Top 0.406: IC7.3 39.37,219.73 40.64,218.46 114.94,218.46 123.19,226.72 IC1.2
ANALOG_A
  Bottom 0.406: IC7.11 46.99,227.35 45.72,226.08 45.72,212.75 47.62,210.84 96.52,210.84 118.75,188.62 127.64,188.62 131.44,184.81 131.44,180.36 133.35,178.46 142.24,178.46 144.15,180.36 144.15,182.27 142.88,183.53 IC1.19
ANALOG_B
  Bottom 0.406: IC1.20 134.62,181 133.35,182.27 133.35,184.81 128.27,189.89 119.38,189.89 97.16,212.11 51.44,212.11 48.26,215.28 48.26,226.08 49.53,227.35 IC7.10
ANALOG_C
  Bottom 0.406: IC7.9 54.61,229.89 55.88,228.62 55.88,214.65 57.15,213.38 97.79,213.38 120.02,191.16 128.91,191.16 132.72,187.34 146.69,187.34 151.76,181 IC1.21
B1.1
  Bottom 0.406: B1.B.MB.4 8.89,234.97 11.43,232.43 IC5.7
B1.2
  Bottom 0.406: B1.B.MB.3 11.43,234.97 13.97,232.43 IC5.6
B1.3
  Bottom 0.406: B1.B.MB.2 13.97,234.97 16.51,232.43 IC5.5
B1.4
  Bottom 0.406: B1.B.MB.1 16.51,234.97 19.05,232.43 IC5.4
B2.1
  Bottom 0.406: IC5.13 19.05,226.08 20.32,227.35 B2.B.MB.4
B2.2
  Bottom 0.406: B2.B.MB.3 22.86,227.35 21.59,226.08 IC5.14
B2.3
  Bottom 0.406: IC5.15 24.13,226.08 25.4,227.35 B2.B.MB.2
B2.4
  Bottom 0.406: IC5.1 26.67,233.7 27.94,234.97 B2.B.MB.1
B3.1
  Bottom 0.406: IC6.7 29.21,191.79 31.75,189.25 PCB3_MB.3
B3.2
  Bottom 0.406: IC6.6 26.67,191.79 29.21,189.25 PCB3_MB.4
B3.3
  Bottom 0.406: IC6.5 24.13,191.79 26.67,189.25 PCB3_MB.5
B3.4
  Bottom 0.406: IC6.4 21.59,191.79 24.13,189.25 PCB3_MB.6
B3.5
  Bottom 0.406: PCB3_MB.7 21.59,189.25 20.32,190.52 20.32,197.5 21.59,198.78 IC6.13
B3.6
  Bottom 0.406: PCB3_MB.8 19.05,189.25 17.78,190.52 17.78,197.5 19.05,198.78 IC6.14
B3.7
  Bottom 0.406: PCB3_MB.9 16.51,189.25 15.24,190.52 15.24,197.5 16.51,198.78 IC6.15
B3.8
  Bottom 0.406: PCB3_MB.10 IC6.1
B5.1
  Bottom 0.406: PCB5_MB.8 88.9,188.62 86.36,191.16 IC3.7
B5.2
  Bottom 0.406: PCB5_MB.7 86.36,188.62 83.82,191.16 IC3.6
B5.3
  Bottom 0.406: PCB5_MB.6 83.82,188.62 81.28,191.16 IC3.5
B5.4
  Bottom 0.406: PCB5_MB.5 81.28,188.62 78.74,191.16 IC3.4
B5.5
  Bottom 0.406: IC3.13 78.74,198.78 77.47,197.5 77.47,189.89 78.74,188.62 PCB5_MB.4
B5.6
  Bottom 0.406: IC3.14 76.2,198.78 74.93,197.5 74.93,189.89 76.2,188.62 PCB5_MB.3
B6.1
  Bottom 0.406: IC4.7 55.88,191.16 58.42,188.62 B6.B.MB.6
B6.2
  Bottom 0.406: IC4.6 53.34,191.16 55.88,188.62 B6.B.MB.5
B6.3
  Bottom 0.406: IC4.5 50.8,191.16 53.34,188.62 B6.B.MB.4
B6.4
  Bottom 0.406: IC4.4 48.26,191.16 50.8,188.62 B6.B.MB.3
B6.5
  Bottom 0.406: B6.B.MB.2 48.26,188.62 46.99,189.89 46.99,197.5 48.26,198.78 IC4.13
B6.6
  Bottom 0.406: B6.B.MB.1 45.72,188.62 44.45,189.89 44.45,197.5 45.72,198.78 IC4.14
B7.1
  Bottom 0.406: IC3.15 73.66,207.03 74.93,208.3 95.25,208.3 116.84,186.71 B7.B.MB.3
B.CUE
  Bottom 0.406: IC4.15 43.18,198.78 41.91,197.5 41.91,184.81 43.81,182.9 96.52,182.9 CUE_MB.4
B.START
  Bottom 0.406: IC4.1 40.64,183.53 43.18,181 106.05,181 106.68,181.63 START_MB.4
B_CLOCK
  Top 0.406: IC6.10 29.21,205.76 | 29.21,205.76 55.88,205.76 | 55.88,205.76 58.42,205.76 60.96,201.95 64.77,201.95 66.67,203.86 86.36,203.86 | 86.36,203.86 104.14,203.86 121.92,221.63 IC1.4 | IC5.10 11.43,212.11 17.78,205.76 29.21,205.76 | IC4.10 55.88,205.76 | 86.36,203.86 IC3.10
B_LOAD
  Top 0.406: IC6.9 31.75,198.78 58.42,198.78 | 58.42,198.78 88.9,198.78 IC3.9 103.5,201.31 121.28,219.09 IC1.5 | IC4.9 58.42,198.78
  Bottom 0.406: IC5.9 8.89,217.19 11.43,214.65 27.3,214.65 31.75,210.21 IC6.9
BUTTONS
  Top 0.406: IC5.12 16.51,218.46 17.78,217.19 115.57,217.19 122.56,224.18 IC1.3
ENC_A
  Bottom 0.406: IC1.38 159.38,224.18 160.66,225.44 ENC_MB.3
ENC_A_
  Bottom 0.406: ENC.4 260.2,192.69 258.93,193.96 251.31,193.96 | ENC01.A 251.22,197.77 251.22,194.05 251.31,193.96 | R6.2 251.31,193.96
ENC_B
  Bottom 0.406: IC1.37 159.38,221.63 160.66,222.91 ENC_MB.4
ENC_B_
  Bottom 0.406: ENC.5 263.37,197.77 261.47,199.68 246.23,199.68 | ENC01.B 246.01,199.46 246.23,199.68 | 246.23,199.68 234.16,199.68 232.26,197.77 R5.2
ENC_SW
  Bottom 0.406: IC1.36 159.38,219.09 160.66,220.37 ENC_MB.5
ENC_SW_
  Bottom 0.406: ENC.3 260.2,190.15 253.98,183.93 ENC01.SW1 251.09,180.21 R7.2
FX1
  Bottom 0.406: FX_MB.1 34.29,234.97 36.83,232.43 IC7.15
FX2
  Bottom 0.406: FX_MB.2 36.83,234.97 39.37,232.43 IC7.14
FX3
  Bottom 0.406: FX_MB.3 39.37,234.97 41.91,232.43 IC7.13
FX4
  Bottom 0.406: FX_MB.4 41.91,234.97 44.45,232.43 IC7.12
GND  (via drill 0.6)  (10 unrouted)
  Top 0.406: IC11.8 92.71,227.35 95.25,224.81 101.6,224.81 102.87,223.54 IC11.13 | 52.07,226.08 59.69,226.08 | 59.69,226.08 IC10.8 | IC10.13 69.85,224.81 68.58,226.08 59.69,226.08 | IC7.8 52.07,226.08 | 52.07,226.08 46.99,226.08 | 46.99,226.08 15.24,226.08 13.97,227.35 8.89,227.35 | 8.89,227.35 6.99,227.35 5.08,225.44 5.08,214.65 15.24,204.49 15.24,191.79 16.51,190.52 31.75,190.52 | IC6.8 31.75,190.52 | IC4.8 58.42,190.52 | 58.42,190.52 88.9,190.52 | 88.9,190.52 IC3.8 | 31.75,190.52 58.42,190.52 | 88.9,190.52 101.6,190.52 104.14,187.98 129.54,187.98 | C3.1 130.81,189.25 129.54,187.98 | PITCH.MB.1 129.54,187.98 | IC5.8 8.89,227.35 | IC7.6 46.99,226.08
  Bottom 0.406: IC7.7 IC7.8 | C3.1 132.72,189.25 126.36,195.6 C1.1 C2.1 126.36,200.68 127,201.31 IC1.12 146.05,201.31 151.13,206.4 IC1.31 157.48,206.4 161.29,210.21 | J1.M2 152.4,243.86 | 152.4,243.86 J1.M1 | J1.4 152.4,241.15 152.4,243.86 | B5.6.P$2 B5.1.P$1 | 23.7,132.96 B5.3.P$2 | 17.17,301.58 BL1.1.C 19.07,301.56 | 19.07,301.56 19.07,306.47 BL1.1.2 | 47.01,301.58 BL1.2.C 19.07,301.56 | BL1.3.C 78.77,301.56 | 78.77,301.56 BL1.4.C | BL1.3.2 80.38,310.81 78.77,309.2 78.77,301.56 | BL6.6.C 204.1,149.19 205.05,150.14 205.05,156.49 | 205.05,156.49 205.05,156.85 BL6.6.2 | BL6.5.2 215.26,158.44 213.3,156.49 205.05,156.49
  other vias: 4.45,181.63 4.45,233.06 48.26,243.23 95.25,243.86 141.6,237.51 119.38,200.05
  pour Top (isolate 0.813): 0.64,247.67 0.64,177.19 173.99,177.19 173.99,247.67
  pour Bottom (isolate 0.813): 0.64,247.67 0.64,177.19 173.99,177.19 173.99,247.67
  pour Bottom (isolate 0.813): 0.66,294.41 0.66,250.6 126.39,250.6 126.39,294.41
  pour Bottom (isolate 0.813): 0.66,345.78 1.29,297.52 127.02,297.52 126.39,345.78
  pour Bottom (isolate 0.813): 0.99,150.89 0.99,101.99 77.82,101.99 77.82,150.89
  pour Bottom (isolate 0.813): 267.82,176.82 267.82,202.58 arc4 229.08,202.58 229.08,176.82
  pour Bottom (isolate 0.813): 135.2,151.41 135.22,101.94 195.52,101.88 195.52,141.25 224.73,141.25 224.73,248.56 180.28,248.56 180.28,151.41
  pour Bottom (isolate 0.813): 190.24,0.83 190.24,23.69 151.51,23.69 151.51,0.83
  pour Bottom (isolate 0.813): 77.05,79.37 134.1,79.37 134.1,0.63 77.05,0.63
  pour Bottom (isolate 0.813): 35.06,47.13 35.06,87.04 0.77,87.04 0.77,47.13
  pour Bottom (isolate 0.813): 34.97,1.13 34.97,41.04 0.68,41.04 0.68,1.13
HDD_A_CPU
  Bottom 0.406: IC1.35 160.02,216.56 161.29,217.83 HDD_OUT_CPU.1
HDD_B_CPU
  Bottom 0.406: IC1.34 160.02,214.02 161.29,215.28 HDD_OUT_CPU.2
L1.1
  Top 0.406: IC10.15 74.93,224.81 76.2,226.08 80.01,226.08 88.9,234.97 B1.L.MB.6
L1.2
  Bottom 0.406: IC10.1 83.82,229.89 86.36,232.43 B1.L.MB.5
L1.3
  Bottom 0.406: IC10.2 74.93,231.16 76.2,232.43 82.55,232.43 83.82,233.7 B1.L.MB.4
L1.4
  Bottom 0.406: IC10.3 72.39,231.16 74.93,233.7 80.01,233.7 81.28,234.97 B1.L.MB.3
L2.1
  Bottom 0.406: IC10.4 69.85,232.43 72.39,234.97 B2.L.MB.6
L2.2
  Bottom 0.406: IC10.5 67.31,232.43 69.85,234.97 B2.L.MB.5
L2.3
  Bottom 0.406: IC10.6 64.77,232.43 67.31,234.97 B2.L.MB.4
L2.4
  Bottom 0.406: IC10.7 62.23,232.43 64.77,234.97 B2.L.MB.3
L6.1
  Bottom 0.406: IC11.15 107.95,224.81 109.22,226.08 111.76,226.08 113.03,227.35 113.03,232.43 110.49,234.97 B6.L.MB.8
L6.2
  Bottom 0.406: B6.L.MB.7 107.95,234.97 110.49,232.43 IC11.1
L6.3
  Bottom 0.406: B6.L.MB.6 105.41,234.97 107.95,232.43 IC11.2
L6.4
  Bottom 0.406: IC11.3 105.41,232.43 102.87,234.97 B6.L.MB.5
L6.5
  Bottom 0.406: B6.L.MB.4 100.33,234.97 102.87,232.43 IC11.4
L6.6
  Bottom 0.406: IC11.5 100.33,232.43 97.79,234.97 B6.L.MB.3
L.CUE  (via drill 0.6 pad 1.93)  (1 unrouted)
  Top 0.406: v83.82,222.27 83.82,227.35 90.81,234.34 95.89,234.34 97.79,232.43 IC11.6
  Bottom 0.406: CUE_MB.3 99.06,197.5 92.71,203.86 86.36,203.86 v83.82,206.4
L.START  (via drill 0.6 pad 1.93)  (1 unrouted)
  Top 0.406: IC11.7 95.25,231.16 93.98,232.43 91.44,232.43 87,227.99 v87,222.27
  Bottom 0.406: START_MB.3 109.22,192.43 95.25,206.4 v87,206.4
LED-CLOCK
  Bottom 0.406: IC11.11 97.79,220.37 97.16,219.73 92.08,219.73 90.81,221 90.81,223.54 88.9,225.44 66.04,225.44 64.77,224.18 IC10.11 64.77,217.19 66.04,215.92 134.62,215.92 139.06,211.48 IC1.8
LED-DATA
  Bottom 0.406: IC10.14 72.39,218.46 73.66,217.19 135.25,217.19 138.43,214.02 IC1.7
LED-LATCH
  Bottom 0.406: IC10.12 67.31,223.54 67.94,224.18 88.27,224.18 89.53,222.91 89.53,220.37 91.44,218.46 100.33,218.46 | 100.33,218.46 135.89,218.46 137.79,216.56 IC1.6 | IC11.12 100.33,218.46
LED-RESET
  Bottom 0.406: IC11.10 95.25,225.44 93.98,226.72 63.5,226.72 62.23,225.44 IC10.10 62.23,215.92 63.5,214.65 133.99,214.65 139.7,208.94 IC1.9
LED.SER
  Bottom 0.406: IC10.9 59.69,226.72 60.96,227.99 104.14,227.99 105.41,226.72 IC11.14
MCLR
  Bottom 0.406: ICSP.5 134.62,231.16 136.53,229.25 IC1.1
N$1
  Top 0.406: IC5.11 13.97,224.81 12.7,226.08 7.62,226.08 6.35,224.81 6.35,215.28 17.78,203.86 17.78,198.78 19.05,197.5 IC6.3
N$2
  Bottom 0.406: R56.1 19.1,32.79 19.1,27.7 19.12,27.67
N$3
  Bottom 0.406: R52.1 12.2,79.42 10.93,80.69 T1.B
N$4
  Bottom 0.406: CUE.3 26.72,34.06 R26.2
N$5
  Bottom 0.406: C3.2 139.06,186.08 IC1.18
N$6
  Bottom 0.406: START.3 26.8,80.06 R52.2
N$7
  Bottom 0.406: R1.1 100.17,26.67 102.08,28.57 SL2.3
N$8
  Bottom 0.406: R3.1 107.8,15.71 | 107.8,15.71 107.8,16.5 109.7,18.41 IC2.3 | R1.2 100.17,15.07 100.81,15.71 107.8,15.71
N$9
  Bottom 0.406: IC2.5 110.97,13.33 109.7,12.06 103.98,12.06 | 103.98,12.06 R2.2 103.98,12.69 | R4.1 102.08,8.25 103.98,10.16 103.98,12.06
N$10
  Bottom 0.406: R2.1 103.98,25.4 105.89,27.3 SL2.2
N$12
  Bottom 0.406: R3.2 IC2.1 113.51,24.76 114.78,26.03 128.12,26.03 132.56,21.59 132.56,12.06 131.93,11.43 HDD_OUT.4
N$13
  Bottom 0.406: R4.2 IC2.7 113.51,6.98 114.78,5.71 121.77,5.71 124.31,8.25 124.31,12.06 126.21,13.97 HDD_OUT.3
N$17
  Top 0.406: IC6.11 26.67,198.14 27.94,196.87 44.45,196.87 45.72,195.6 IC4.3
N$18
  Bottom 0.406: IC3.3 76.2,189.89 77.47,188.62 77.47,184.81 76.83,184.17 69.85,184.17 68.58,185.44 68.58,194.97 66.04,197.5 54.61,197.5 53.34,198.78 IC4.11
N$19  (via drill 0.6 pad 3.81)
  other vias: 122,193.71
N$20
  Bottom 0.406: B7.B.3 162.86,18.68 B7.1.P$2 168.33,17.66 169.92,16.07 178.82,16.07 180.09,17.34 R53.1
N$21
  Bottom 0.406: R28.1 184.73,106.32 191.08,112.67 B6.L.8
N$22
  Bottom 0.406: B6.B.5 146.63,124.74 147.9,123.47 R33.1 151.79,121.56 157.43,115.93 169.49,115.93 170.96,117.4 BL6.2.4
N$23
  Bottom 0.406: R48.1 67.33,300.31 111.78,300.31 121.94,310.47 B1.L.6
N$24
  Bottom 0.406: CUE.4 24.81,31.52 | 24.81,31.52 17.83,38.5 R51.2 | ARC01.P$1 14.04,18.84 24.81,29.61 24.81,31.52
N$25
  Bottom 0.406: BL6.3.4 150.44,138.96 150.44,139.98 149.8,140.61 145.99,140.61 145.36,139.98 R34.1 145.36,131.72 143.45,129.82 B6.B.3
N$26
  Bottom 0.406: START.4 24.9,77.52 | 24.9,77.52 17.91,84.5 R54.2 | ARC02.P$1 13.97,64.69 24.9,75.61 24.9,77.52
N$27
  Bottom 0.406: R44.1 7.39,305.01 13.36,297.77 121.31,297.77 125.75,302.21 125.75,319.36 125.12,319.99 B1.L.4
N$28
  Bottom 0.406: B2.L.5 194.25,194.59 R40.1
N$29
  Bottom 0.406: D1.A 149.22,237.51 150.87,239.15 J1.1
N$30
  Bottom 0.406: B6.B.4 145.99,127.28 147.9,129.18 147.9,136.17 | R11.1 147.9,136.17 | 147.9,136.17 168.68,136.17 BL6.4.4
N$31
  Bottom 0.406: B6.B.2 142.82,132.36 144.09,133.63 144.09,143.15 145.99,145.06 179.73,145.06 180.28,144.5 192.35,144.5 193.62,145.78 R27.1 205.6,147.6 211.45,153.44 BL6.5.4
N$32
  Bottom 0.406: FX.3 10.82,330.79 13.99,333.96 73.05,333.96 77.02,337.94 P3.P$1
N$33
  Bottom 0.406: R30.1 168.22,106.32 169.49,105.05 178.38,105.05 180.92,107.59 184.09,107.59 187.9,111.4 187.9,117.75 188.54,118.39 B6.L.7
N$34
  Bottom 0.406: BL6.6.4 196.92,153.44 R29.1 191,147.68 189.18,147.68 186.63,150.22 184.09,150.22 179.57,146.33 145.36,146.33 142.18,143.15 142.18,134.9 B6.B.1
N$35
  Bottom 0.406: B6.B.6 144.72,122.2 R32.1 147.84,118.44 BL6.1.4
N$36
  Bottom 0.406: B6.L.4 188.54,126.01 185.36,129.18 185.36,141.88 186.63,143.15 192.9,143.15 195.53,145.78 213.94,145.78 218.38,149.59 222.83,149.59 222.83,159.03 220.29,161.57 217.75,161.57 216.48,162.84 R9.1
N$37
  Bottom 0.406: R31.1 166.95,126.64 169.49,124.1 183.46,124.1 186.63,120.93 B6.L.6
N$38
  Bottom 0.406: R8.1 184.09,126.64 187.27,123.47 B6.L.5
N$39
  Bottom 0.406: B6.L.3 188.54,128.55 186.63,130.45 186.63,141.25 187.27,141.88 221.56,141.88 224.1,144.42 224.1,164.74 220.92,167.92 202.51,167.92 201.87,167.28 R10.1
N$40
  Bottom 0.406: B2.B.3 220.29,195.86 217.11,199.03 217.11,202.84 215.84,204.11 213.3,204.11 212.03,205.38 R35.1 212.03,206.65 212.67,207.29 215.84,207.29 219.02,210.46 219.02,213 BL2.4.4
N$41
  Bottom 0.406: BL2.3.4 203.46,211.41 201.87,209.83 R37.1 201.87,204.11 203.14,202.84 214.57,202.84 215.84,201.57 215.84,198.4 220.92,193.32 B2.B.2
N$42
  Bottom 0.406: B2.B.4 219.65,198.4 218.38,199.67 218.38,204.11 216.48,206.02 | 216.48,206.02 R39.1 | BL2.2.4 220.99,229.44 222.19,228.24 222.19,211.73 216.48,206.02
N$43
  Bottom 0.406: B2.B.1 219.65,190.78 219.02,191.41 219.02,193.32 213.94,198.4 213.94,200.94 213.3,201.57 201.24,201.57 199.33,203.48 R41.1 199.33,228.88 199.97,229.51 203.39,229.51 BL2.1.4
N$44
  Bottom 0.406: B2.L.6 191.71,197.13 R36.1
N$45
  Bottom 0.406: B2.L.4 195.52,192.05 197.43,193.95 206.32,193.95 206.95,194.59 R38.1
N$46
  Bottom 0.406: B2.L.3 195.52,189.51 198.7,192.68 208.22,192.68 209.49,193.95 R42.1
N$47
  Bottom 0.406: R55.2 19.18,78.79 19.18,73.8 19.05,73.67
N$48
  Bottom 0.406: R46.1 38.12,299.04 112.42,299.04 124.48,311.1 124.48,316.82 123.85,317.45 B1.L.5
N$49
  Bottom 0.406: R26.1 12.11,33.42 10.84,34.69 T2.B
N$50
  Bottom 0.406: R50.1 B1.L.3
N$51
  Bottom 0.406: R49.1 28.6,318.72 | 28.6,318.72 28.6,307.68 26.69,305.77 23.46,305.77 BL1.1.4 | B1.B.1 5.74,317.45 7.01,318.72 28.6,318.72 | 28.6,318.72
N$52
  Bottom 0.406: BL1.2.4 57.21,305.81 59.08,307.68 59.08,314.66 R47.1 57.81,320.63 7.01,320.63 6.38,319.99 B1.B.2
N$53
  Bottom 0.406: FX.4 10.19,328.25 14.63,332.69 100.99,332.69 107.02,338.73 P4.P$1
N$54
  Bottom 0.406: FX.2 11.46,333.33 13.36,335.23 44.48,335.23 47.02,337.78 P2.P$1
N$55
  Bottom 0.406: BL1.3.4 83.15,305.77 87.02,305.77 88.92,307.68 R45.1 88.92,321.26 88.29,321.9 7.01,321.9 6.38,322.53 B1.B.3
N$56
  Bottom 0.406: BL1.4.4 114.75,305.81 116.86,307.93 R43.1 116.86,318.09 115.59,319.36 94.64,319.36 90.83,323.17 7.64,323.17 5.74,325.07 B1.B.4
N$57
  Bottom 0.406: FX.1 11.46,335.87 16.39,340.8 P1.P$1
N$58
  Bottom 0.406: PCB3.7 29.23,286.15 26.23,289.15 B3.5.P$2 20.17,289.15 17.8,286.79 R12.1
N$59
  Bottom 0.406: T2.C 8.94,30.24 11.5,27.67
N$60
  Bottom 0.406: T1.C 9.02,76.08 11.43,73.67
N$61
  Bottom 0.406: PCB3.8 31.77,290.6 33.68,292.5 111.15,292.5 113.06,290.6 113.06,289.48 B3.3.P$2 117.22,289.15 R13.1
N$62
  Bottom 0.406: PCB3.9 34.31,289.33 36.22,291.24 81.31,291.24 83.21,289.33 83.21,289.32 B3.1.P$2 87.37,289.15 R14.1
N$63  (via drill 0.6 pad 3.81)
  other vias: 122,205.31
N$64  (via drill 0.6 pad 3.81)
  other vias: 135,205.31
N$65
  Bottom 0.406: R15.1 57.52,289.15 B3.7.P$2 46.03,289.15 43.84,286.97 43.84,283.15 36.85,276.17 PCB3.10
N$66
  Bottom 0.406: B5.2.P$2 46.3,137.96 49.25,135.01 49.25,128.66 51.15,126.76 R20.1 60.04,142 58.95,143.09 PCB5.5
N$67
  Bottom 0.406: B3.8.P$2 56.4,269.15 57.81,267.74 R17.1 57.81,258.39 54,254.58 24.79,254.58 24.16,255.22 PCB3.5
N$68
  Bottom 0.406: B3.4.P$2 86.24,269.15 87.66,267.74 R18.1 87.66,256.49 84.48,253.31 22.25,253.31 21.61,253.94 PCB3.4
N$69  (1 unrouted)
  Bottom 0.406: R16.1 21.61,274.9 23.52,272.82 23.52,269.01 24.79,269.01 26.7,267.11 PCB3.6
N$70
  Bottom 0.406: B3.2.P$2 116.08,269.15 117.5,267.74 R19.1 117.5,262.84 106.7,252.04 20.34,252.04 19.07,253.31 PCB3.3
N$71
  Bottom 0.406: PCB5.4 56.41,144.54 53.87,142 35.91,142 34.01,140.09 34.01,127.39 30.2,123.58 R24.1 27.02,114.06 25.85,112.88 B5.3.P$1
N$72
  Bottom 0.406: BL6.4.A 177.21,127.38 176.47,126.64 R8.2
N$73
  Bottom 0.406: BL6.5.A 207.73,162.69 206.32,164.11 R9.2
N$74
  Bottom 0.406: BL6.6.A 193.13,162.69 191.71,164.11 R10.2
N$76  (via drill 0.6 pad 3.81)
  other vias: 170,205.31
N$77
  Bottom 0.406: BL2.1.A 196.23,239.67 190.44,239.67 188.54,237.77 188.54,209.19 191.71,206.02 R36.2
N$78
  Bottom 0.406: R38.2 206.95,209.91 210.13,213.09 210.13,222.61 211.4,223.88 211.4,237.85 212.24,238.69 BL2.2.A
N$79
  Bottom 0.406: B5.5.P$1 46.17,112.88 49.25,115.96 49.25,121.68 51.15,123.58 R21.1 61.31,123.58 61.95,124.22 61.95,127.84 61.49,128.3 PCB5.6
N$80  (1 unrouted)
  Bottom 0.406: R22.1 73.38,114.06 72.11,112.79 67.66,112.79 67.57,112.88 67.38,112.88 64.03,116.23 PCB5.7
N$81
  Bottom 0.406: PCB5.8 66.57,139.73 68.33,137.96 B5.1.P$2 68.92,138.19 R23.1
N$82
  Bottom 0.406: R30.2 155.52,106.32 157.21,108.01 BL6.1.A
N$83
  Bottom 0.406: PCB5.3 53.87,144.54 52.6,143.27 28.29,143.27 27.02,142 27.02,137.55 | B5.4.P$2 26.61,137.96 27.02,137.55 | 27.02,137.55 R25.1
N$84
  Bottom 0.406: R40.2 195.52,221.97 196.24,222.69 BL2.3.A
N$85
  Bottom 0.406: BL6.2.A 177.21,107.69 175.84,106.32 R28.2
N$86
  Bottom 0.406: R42.2 209.49,210.54 211.4,212.45 211.4,221.98 212.12,222.69 BL2.4.A
N$89  (via drill 0.6 pad 3.81)
  other vias: 170,243.31
N$90  (via drill 0.6 pad 3.81)
  other vias: 135,243.31
N$91  (via drill 0.6 pad 3.81)
  other vias: 122,243.31
N$92  (via drill 0.6 pad 3.81)
  other vias: 62,243.31
N$93  (via drill 0.6 pad 3.81)
  other vias: 5,243.31
N$94
  Bottom 0.406: R31.2 156.15,126.64 157.21,127.7 BL6.3.A
N$95  (via drill 0.6 pad 3.81)
  other vias: 5,193.71
N$96  (via drill 0.6 pad 3.81)
  other vias: 63,193.71
N$97  (via drill 0.6 pad 3.81)
  other vias: 17.02,328.41
N$98  (via drill 0.6 pad 3.81)
  other vias: 63,205.23
N$99  (via drill 0.6 pad 3.81)
  other vias: 47.02,328.41
N$100  (via drill 0.6 pad 3.81)
  other vias: 77.03,328.41
N$101  (via drill 0.6 pad 3.81)
  other vias: 107.03,328.41
N$102  (via drill 0.6 pad 3.81)
  other vias: 122.03,341.41
N$103  (via drill 0.6 pad 3.81)
  other vias: 122.03,303.41
N$104  (via drill 0.6 pad 3.81)
  other vias: 5.03,341.41
N$105  (via drill 0.6 pad 3.81)
  other vias: 5.03,303.41
N$106  (via drill 0.6 pad 3.81)
  other vias: 5.03,290.05
N$107  (via drill 0.6 pad 3.81)
  other vias: 122.03,290.05
N$108
  Bottom 0.406: BL1.1.A 17.02,315.06 15.27,316.82 R44.2
N$109
  Bottom 0.406: R46.2 36.85,313.01 38.91,315.06 BL1.2.A
N$110
  Bottom 0.406: R48.2 66.06,313.01 68.12,315.06 BL1.3.A
N$111
  Bottom 0.406: BL1.4.A 96.69,315.06 95.91,314.28 R50.2
N$112  (via drill 0.6 pad 3.81)
  other vias: 122.03,255.05
N$113  (via drill 0.6 pad 3.81)
  other vias: 5.03,255.05
N$114  (via drill 0.6 pad 3.81)
  other vias: 5.35,146.42
N$115  (via drill 0.6 pad 3.81)
  other vias: 73.35,146.42
N$116  (via drill 0.6 pad 3.81)
  other vias: 73.35,106.42
N$117  (via drill 0.6 pad 3.81)
  other vias: 5.35,106.42
N$118  (via drill 0.6 pad 3.81)
  other vias: 185.87,5.33
N$119  (via drill 0.6 pad 3.81)
  other vias: 155.87,5.33
N$120  (via drill 0.6 pad 3.81)
  other vias: 155.87,19.33
N$121  (via drill 0.6 pad 3.81)
  other vias: 185.87,19.33
N$122  (via drill 0.6 pad 3.81)
  other vias: 80.42,75
N$123  (via drill 0.6 pad 3.81)
  other vias: 130.41,75
N$124  (via drill 0.6 pad 3.81)
  other vias: 80.42,5
N$125  (via drill 0.6 pad 3.81)
  other vias: 130.41,5
N$126  (via drill 0.6 pad 3.81)
  other vias: 94.07,31.77
N$127  (via drill 0.6 pad 3.81)
  other vias: 129.62,52.11
N$128  (via drill 0.6 pad 3.81)
  other vias: 94.26,72.73
N$129  (via drill 0.6 pad 3.81)
  other vias: 140.22,106.94
N$130  (via drill 0.6 pad 3.81)
  other vias: 140.22,146.94
N$131  (via drill 0.6 pad 3.81)
  other vias: 185.22,146.94
N$132  (via drill 0.6 pad 3.81)
  other vias: 191.22,106.94
N$133  (via drill 0.6 pad 3.81)
  other vias: 220.22,145.94
N$134  (via drill 0.6 pad 3.81)
  other vias: 220.22,164.94
N$135  (via drill 0.6 pad 3.81)
  other vias: 185.2,164.95
N$136  (via drill 0.6 pad 3.81)
  other vias: 185.22,205.94
N$137  (via drill 0.6 pad 3.81)
  other vias: 220.22,205.94
N$138  (via drill 0.6 pad 3.81)
  other vias: 220.22,243.94
N$139  (via drill 0.6 pad 3.81)
  other vias: 185.22,243.94
N$140  (via drill 0.6 pad 3.81)
  other vias: 5,205.31
N$141  (via drill 0.6 pad 1.42)
  other vias: 157.2,140.41
N$142  (via drill 0.6 pad 1.42)
  other vias: 157.21,131.43
N$143  (via drill 0.6 pad 1.42)
  other vias: 177.21,140.43
N$144  (via drill 0.6 pad 1.42)
  other vias: 177.21,131.43
N$145  (via drill 0.6 pad 1.42)
  other vias: 177.21,120.43
N$146  (via drill 0.6 pad 1.42)
  other vias: 157.21,120.43
N$147  (via drill 0.6 pad 1.42)
  other vias: 157.21,111.43
N$148  (via drill 0.6 pad 1.42)
  other vias: 177.21,111.43
N$149  (via drill 0.6 pad 1.42)
  other vias: 213.21,151.44
N$150  (via drill 0.6 pad 1.42)
  other vias: 197.21,151.43
N$151  (via drill 0.6 pad 1.42)
  other vias: 197.21,160.43
N$152  (via drill 0.6 pad 1.42)
  other vias: 213.21,160.44
N$153  (via drill 0.6 pad 1.42)
  other vias: 213.22,211.42
N$154  (via drill 0.6 pad 1.42)
  other vias: 213.21,220.42
N$155  (via drill 0.6 pad 1.42)
  other vias: 197.21,220.43
N$156  (via drill 0.6 pad 1.42)
  other vias: 197.21,211.44
N$157  (via drill 0.6 pad 1.42)
  other vias: 197.21,227.43
N$158  (via drill 0.6 pad 1.42)
  other vias: 197.21,236.43
N$159  (via drill 0.6 pad 1.42)
  other vias: 213.22,236.43
N$160  (via drill 0.6 pad 1.42)
  other vias: 213.21,227.41
N$161  (via drill 0.6 pad 1.42)
  other vias: 17.16,312.8
N$162  (via drill 0.6 pad 1.42)
  other vias: 17.16,303.8
N$163  (via drill 0.6 pad 1.42)
  other vias: 47.02,312.81
N$164  (via drill 0.6 pad 1.42)
  other vias: 47.01,303.8
N$165  (via drill 0.6 pad 1.42)
  other vias: 76.86,312.8
N$166  (via drill 0.6 pad 1.42)
  other vias: 76.86,303.8
N$167  (via drill 0.6 pad 1.42)
  other vias: 107.34,312.8
N$168  (via drill 0.6 pad 1.42)
  other vias: 107.33,303.8
N$169  (via drill 0.6 pad 6.45)
  other vias: 205.21,185.94
N$171  (via drill 0.6 pad 42)
  other vias: 105.91,52.25
OSC1
  Bottom 0.406: IC1.13 Q1.1 C2.2
OSC2
  Bottom 0.406: IC1.14 135.25,196.24 | 135.25,196.24 C1.2 | Q1.2 135.25,196.24
PGC
  Bottom 0.406: IC1.39 151.76,226.72 150.5,225.44 132.72,225.44 129.54,228.62 ICSP.3
PGD
  Bottom 0.406: ICSP.4 132.08,231.8 135.89,227.99 151.76,227.99 153.03,229.25 IC1.40
PITCH
  Bottom 0.406: IC7.5 44.45,212.11 46.99,209.57 95.89,209.57 118.11,187.34 123.19,187.34 124.46,186.08 PITCH.MB.3
USB_D+
  Bottom 0.406: J1.3 165.27,241.15 170.18,236.24 170.18,210.21 167,207.03 167,191.16 164.47,188.62 IC1.24
USB_D-
  Bottom 0.406: J1.2 165.37,239.15 168.91,235.61 168.91,210.84 165.74,207.67 165.74,191.79 163.83,189.89 154.94,189.89 154.31,189.25 154.31,186.71 154.94,186.08 IC1.23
